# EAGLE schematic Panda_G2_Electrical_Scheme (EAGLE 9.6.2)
AUTHOR: Andrea Maroso; TITLE: Electrical Scheme

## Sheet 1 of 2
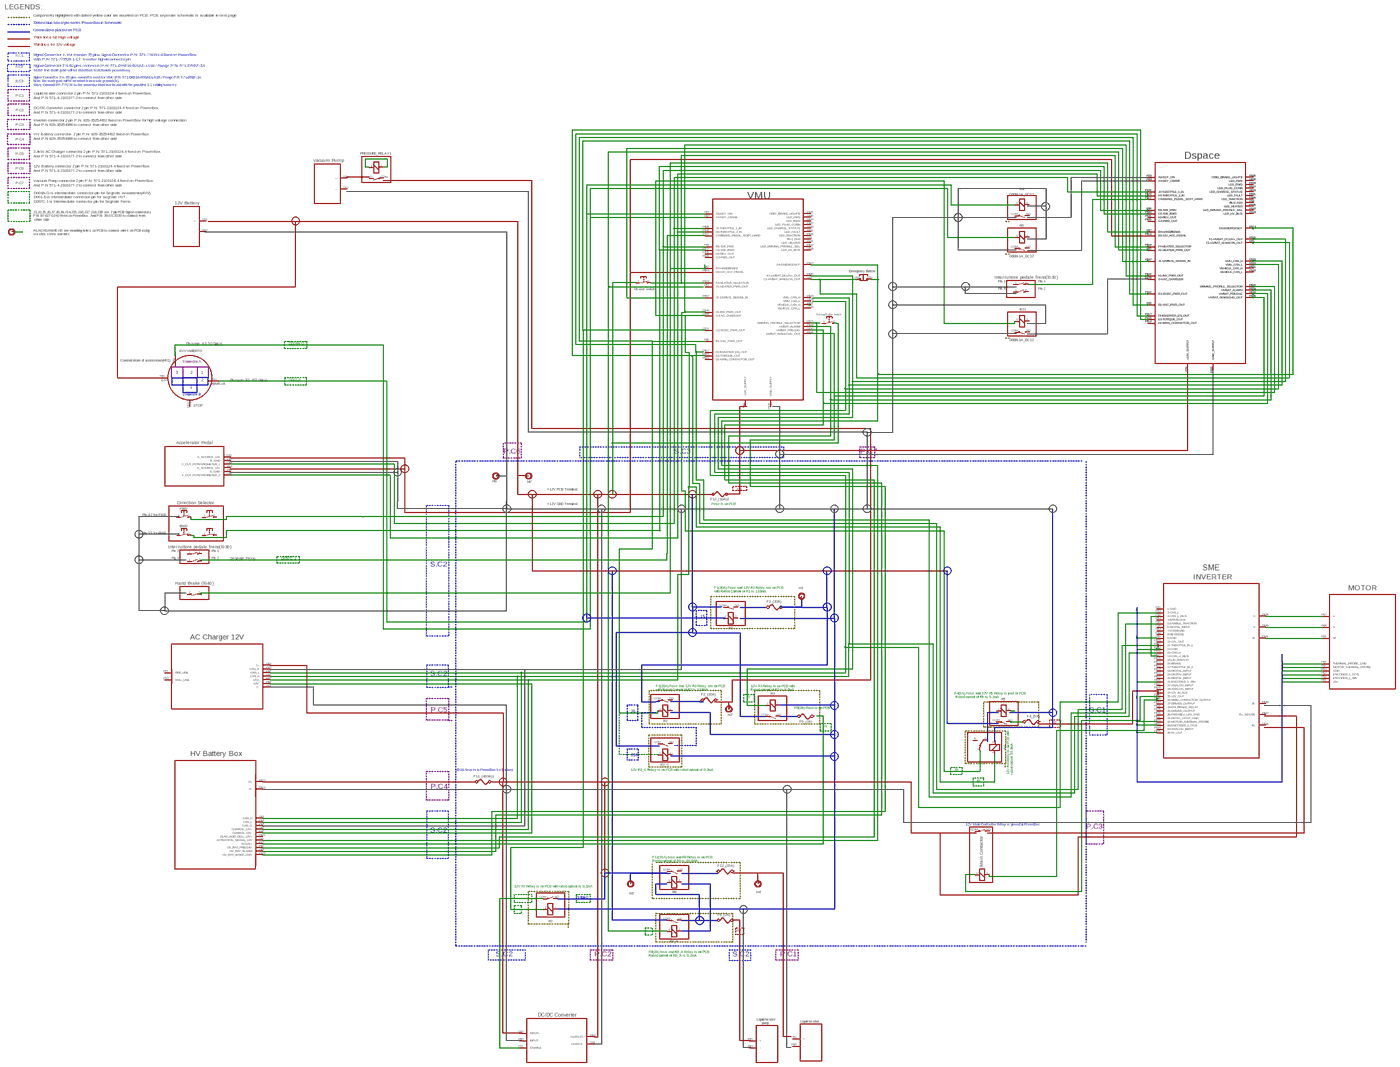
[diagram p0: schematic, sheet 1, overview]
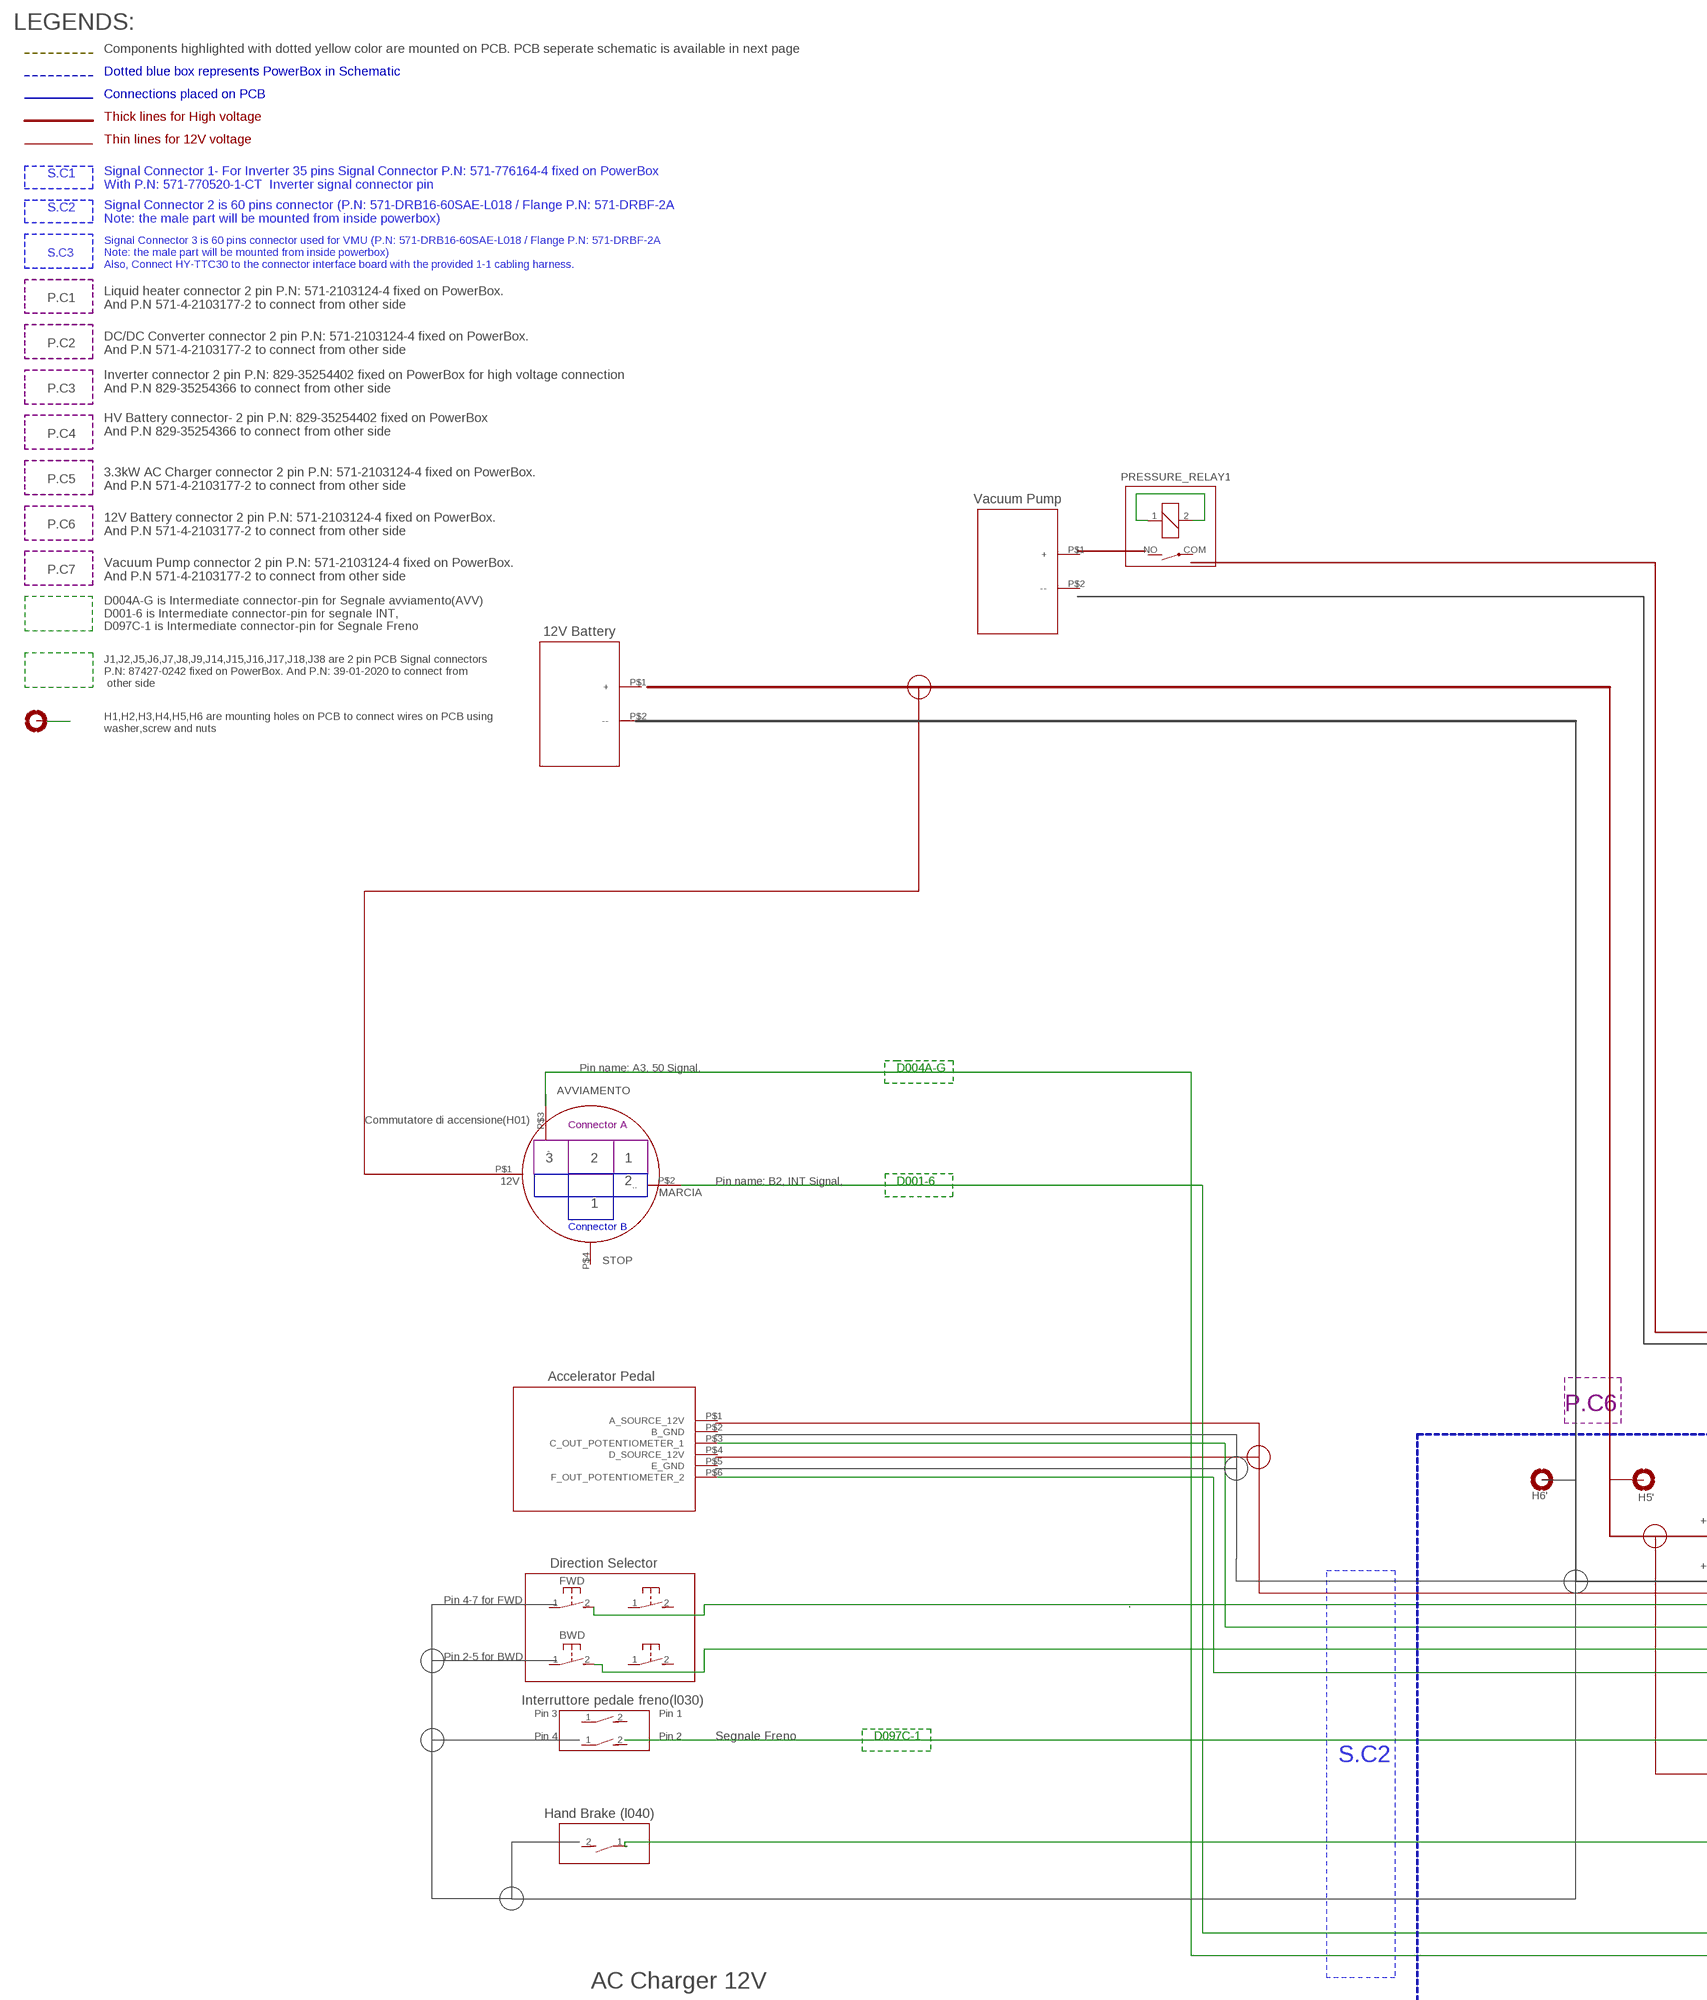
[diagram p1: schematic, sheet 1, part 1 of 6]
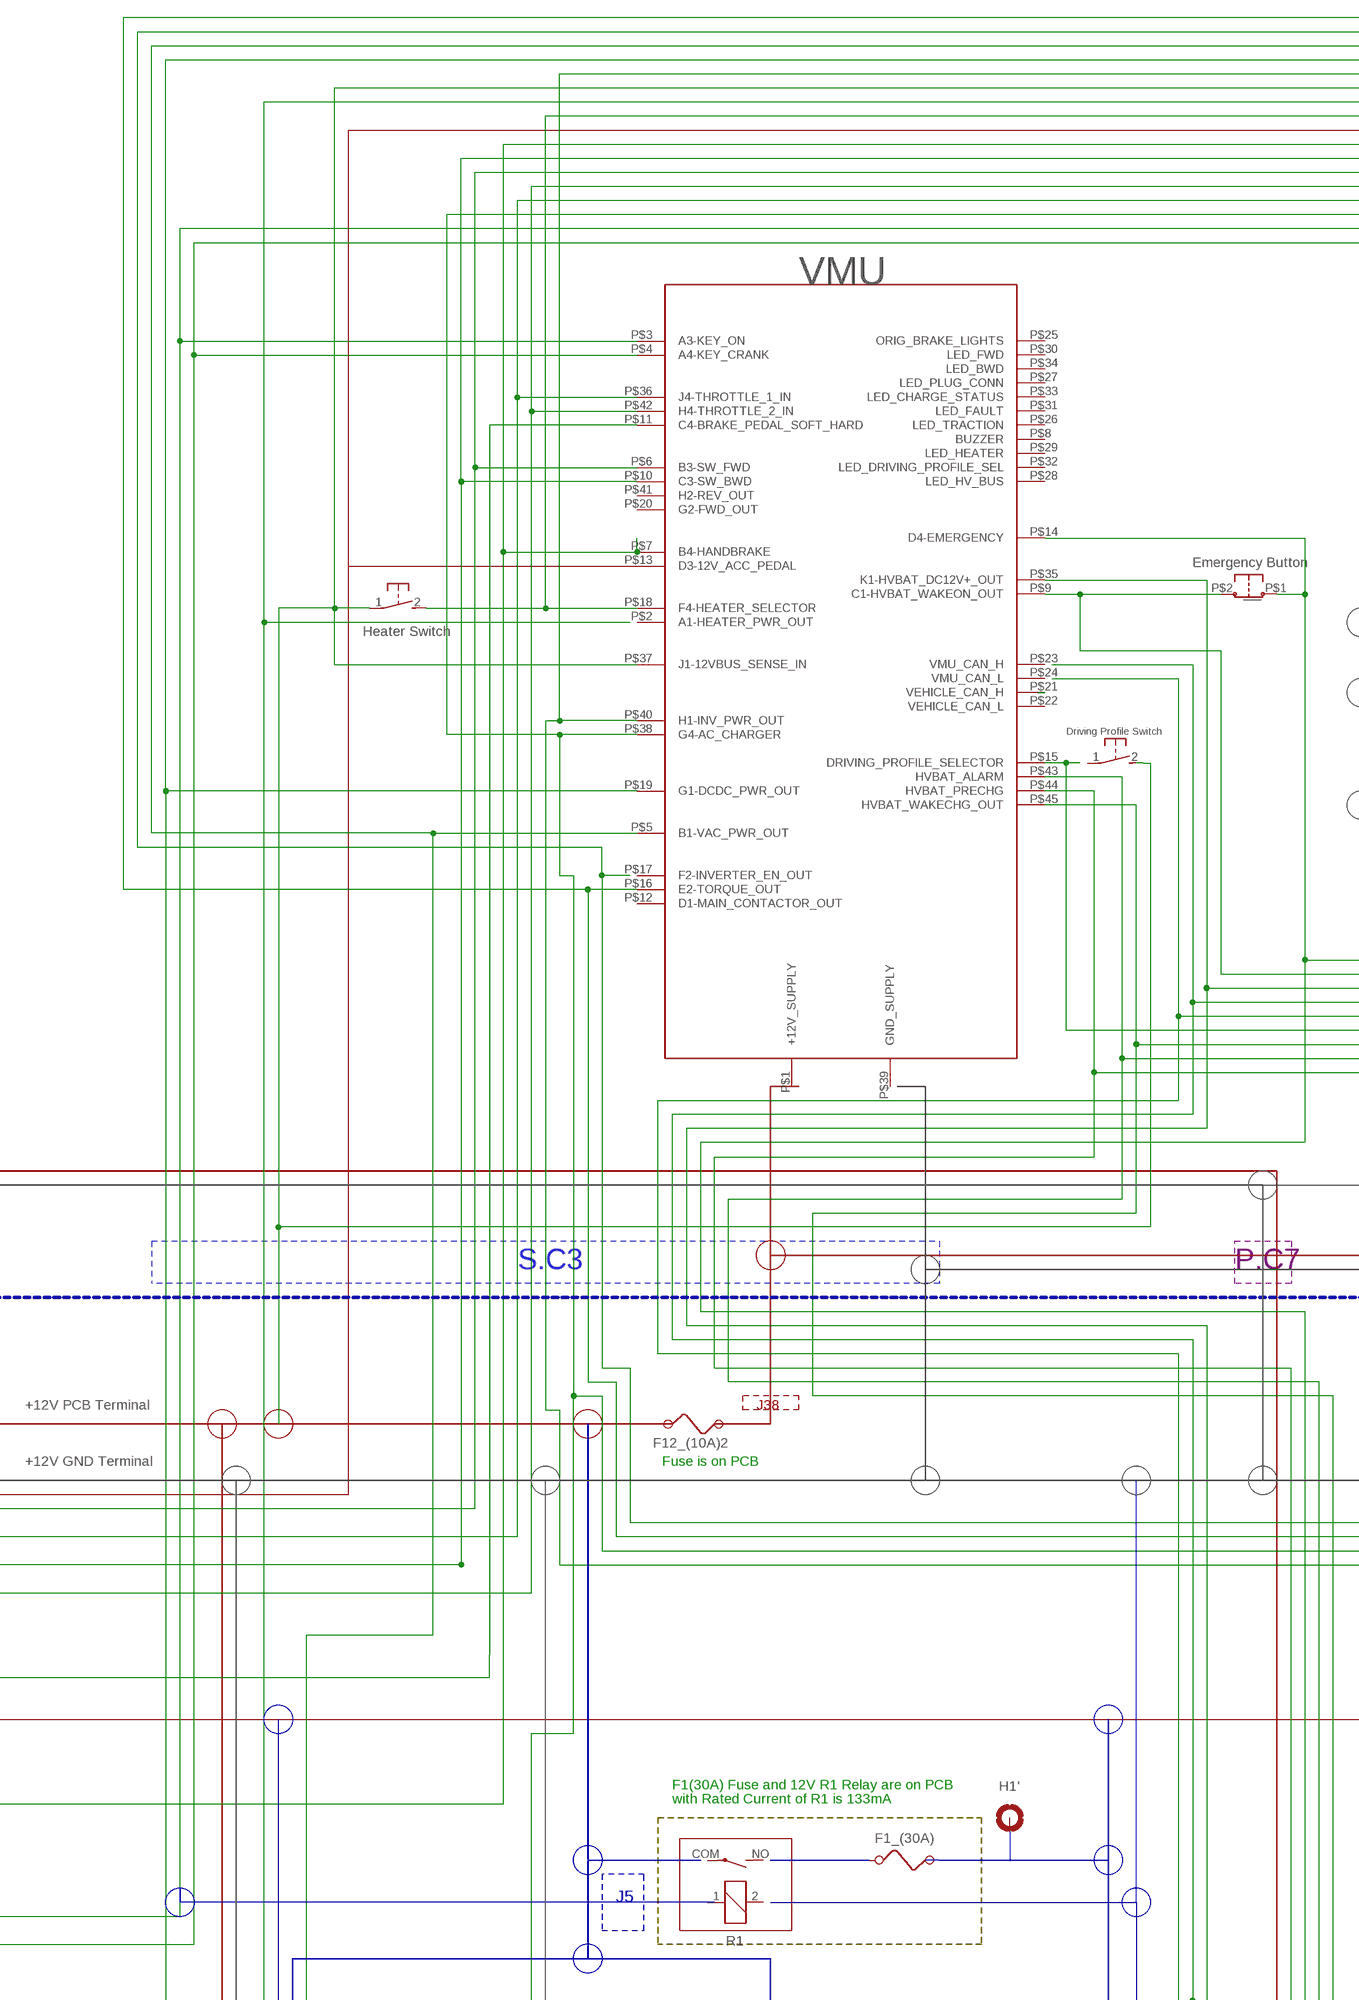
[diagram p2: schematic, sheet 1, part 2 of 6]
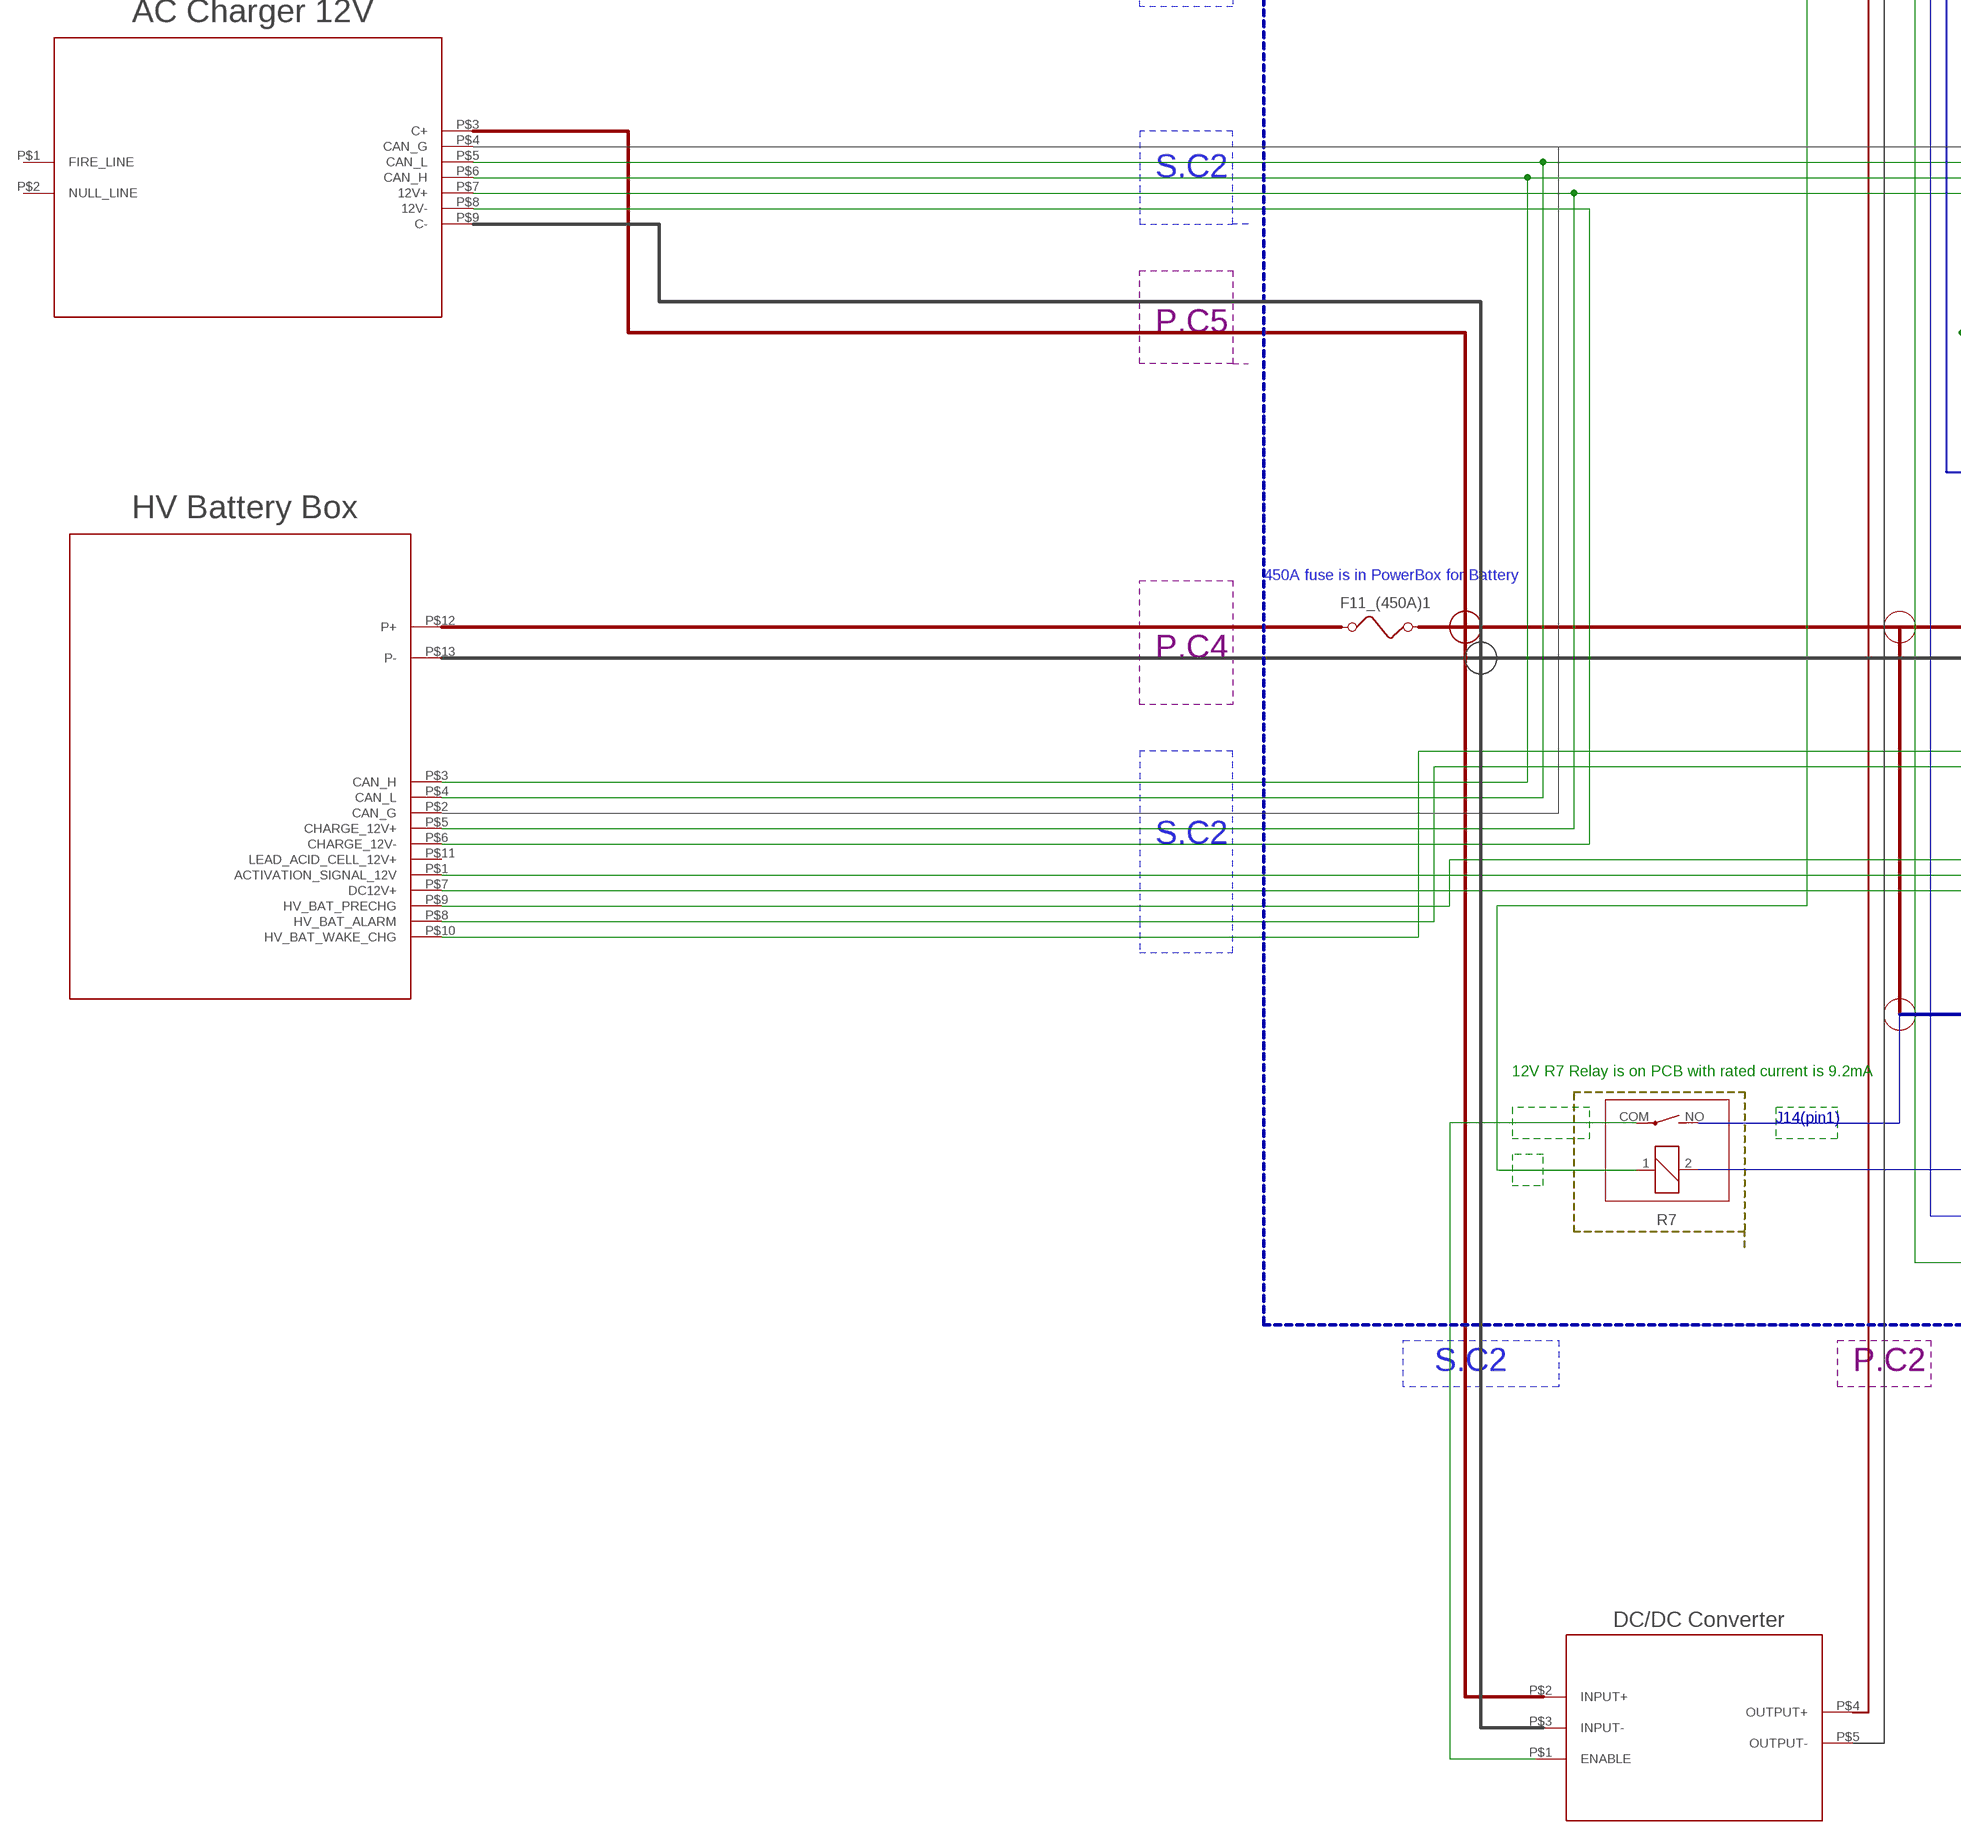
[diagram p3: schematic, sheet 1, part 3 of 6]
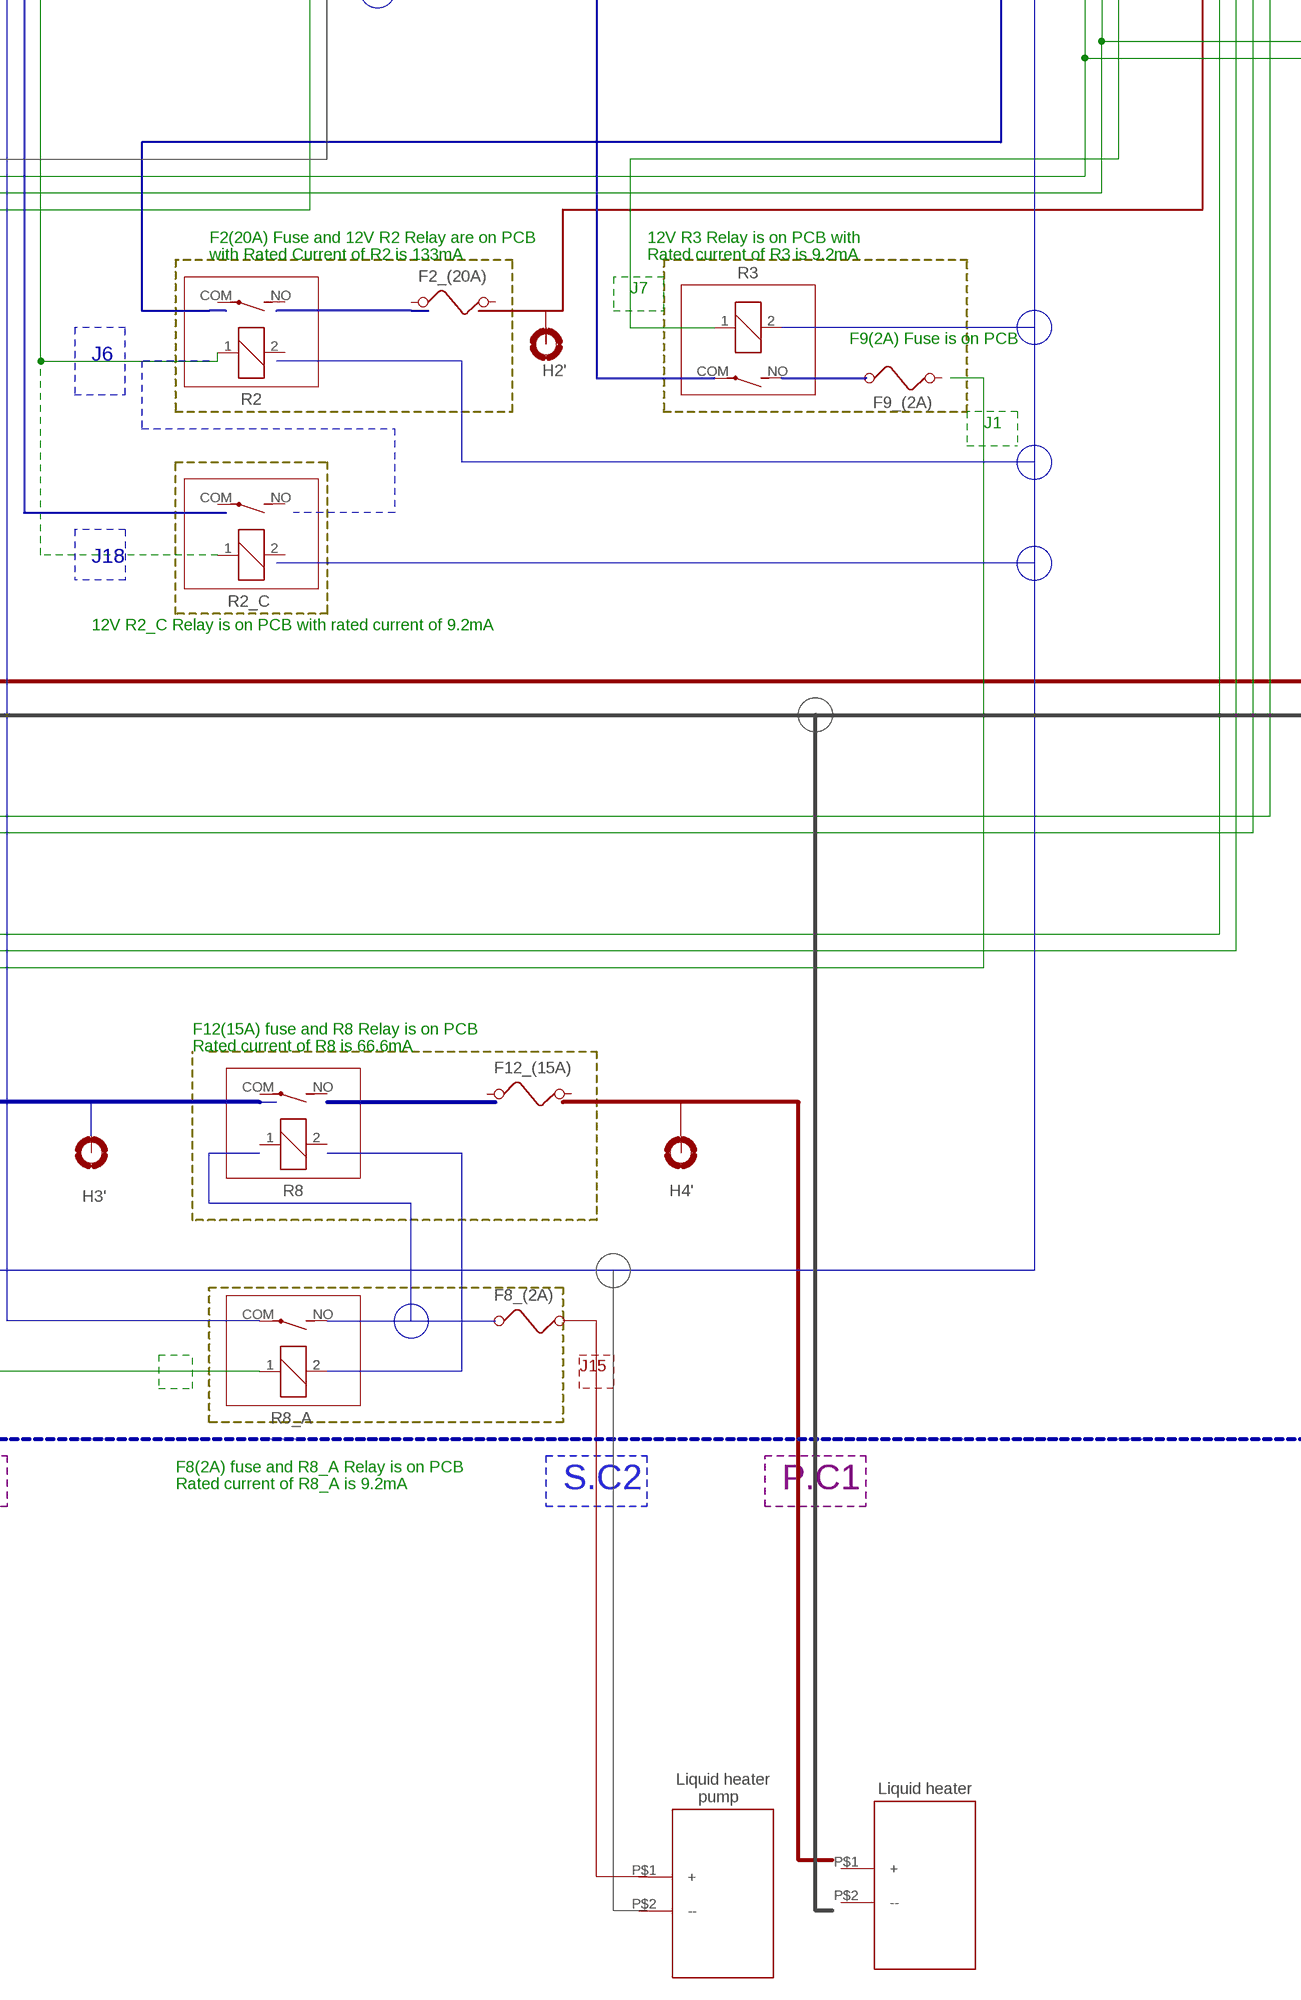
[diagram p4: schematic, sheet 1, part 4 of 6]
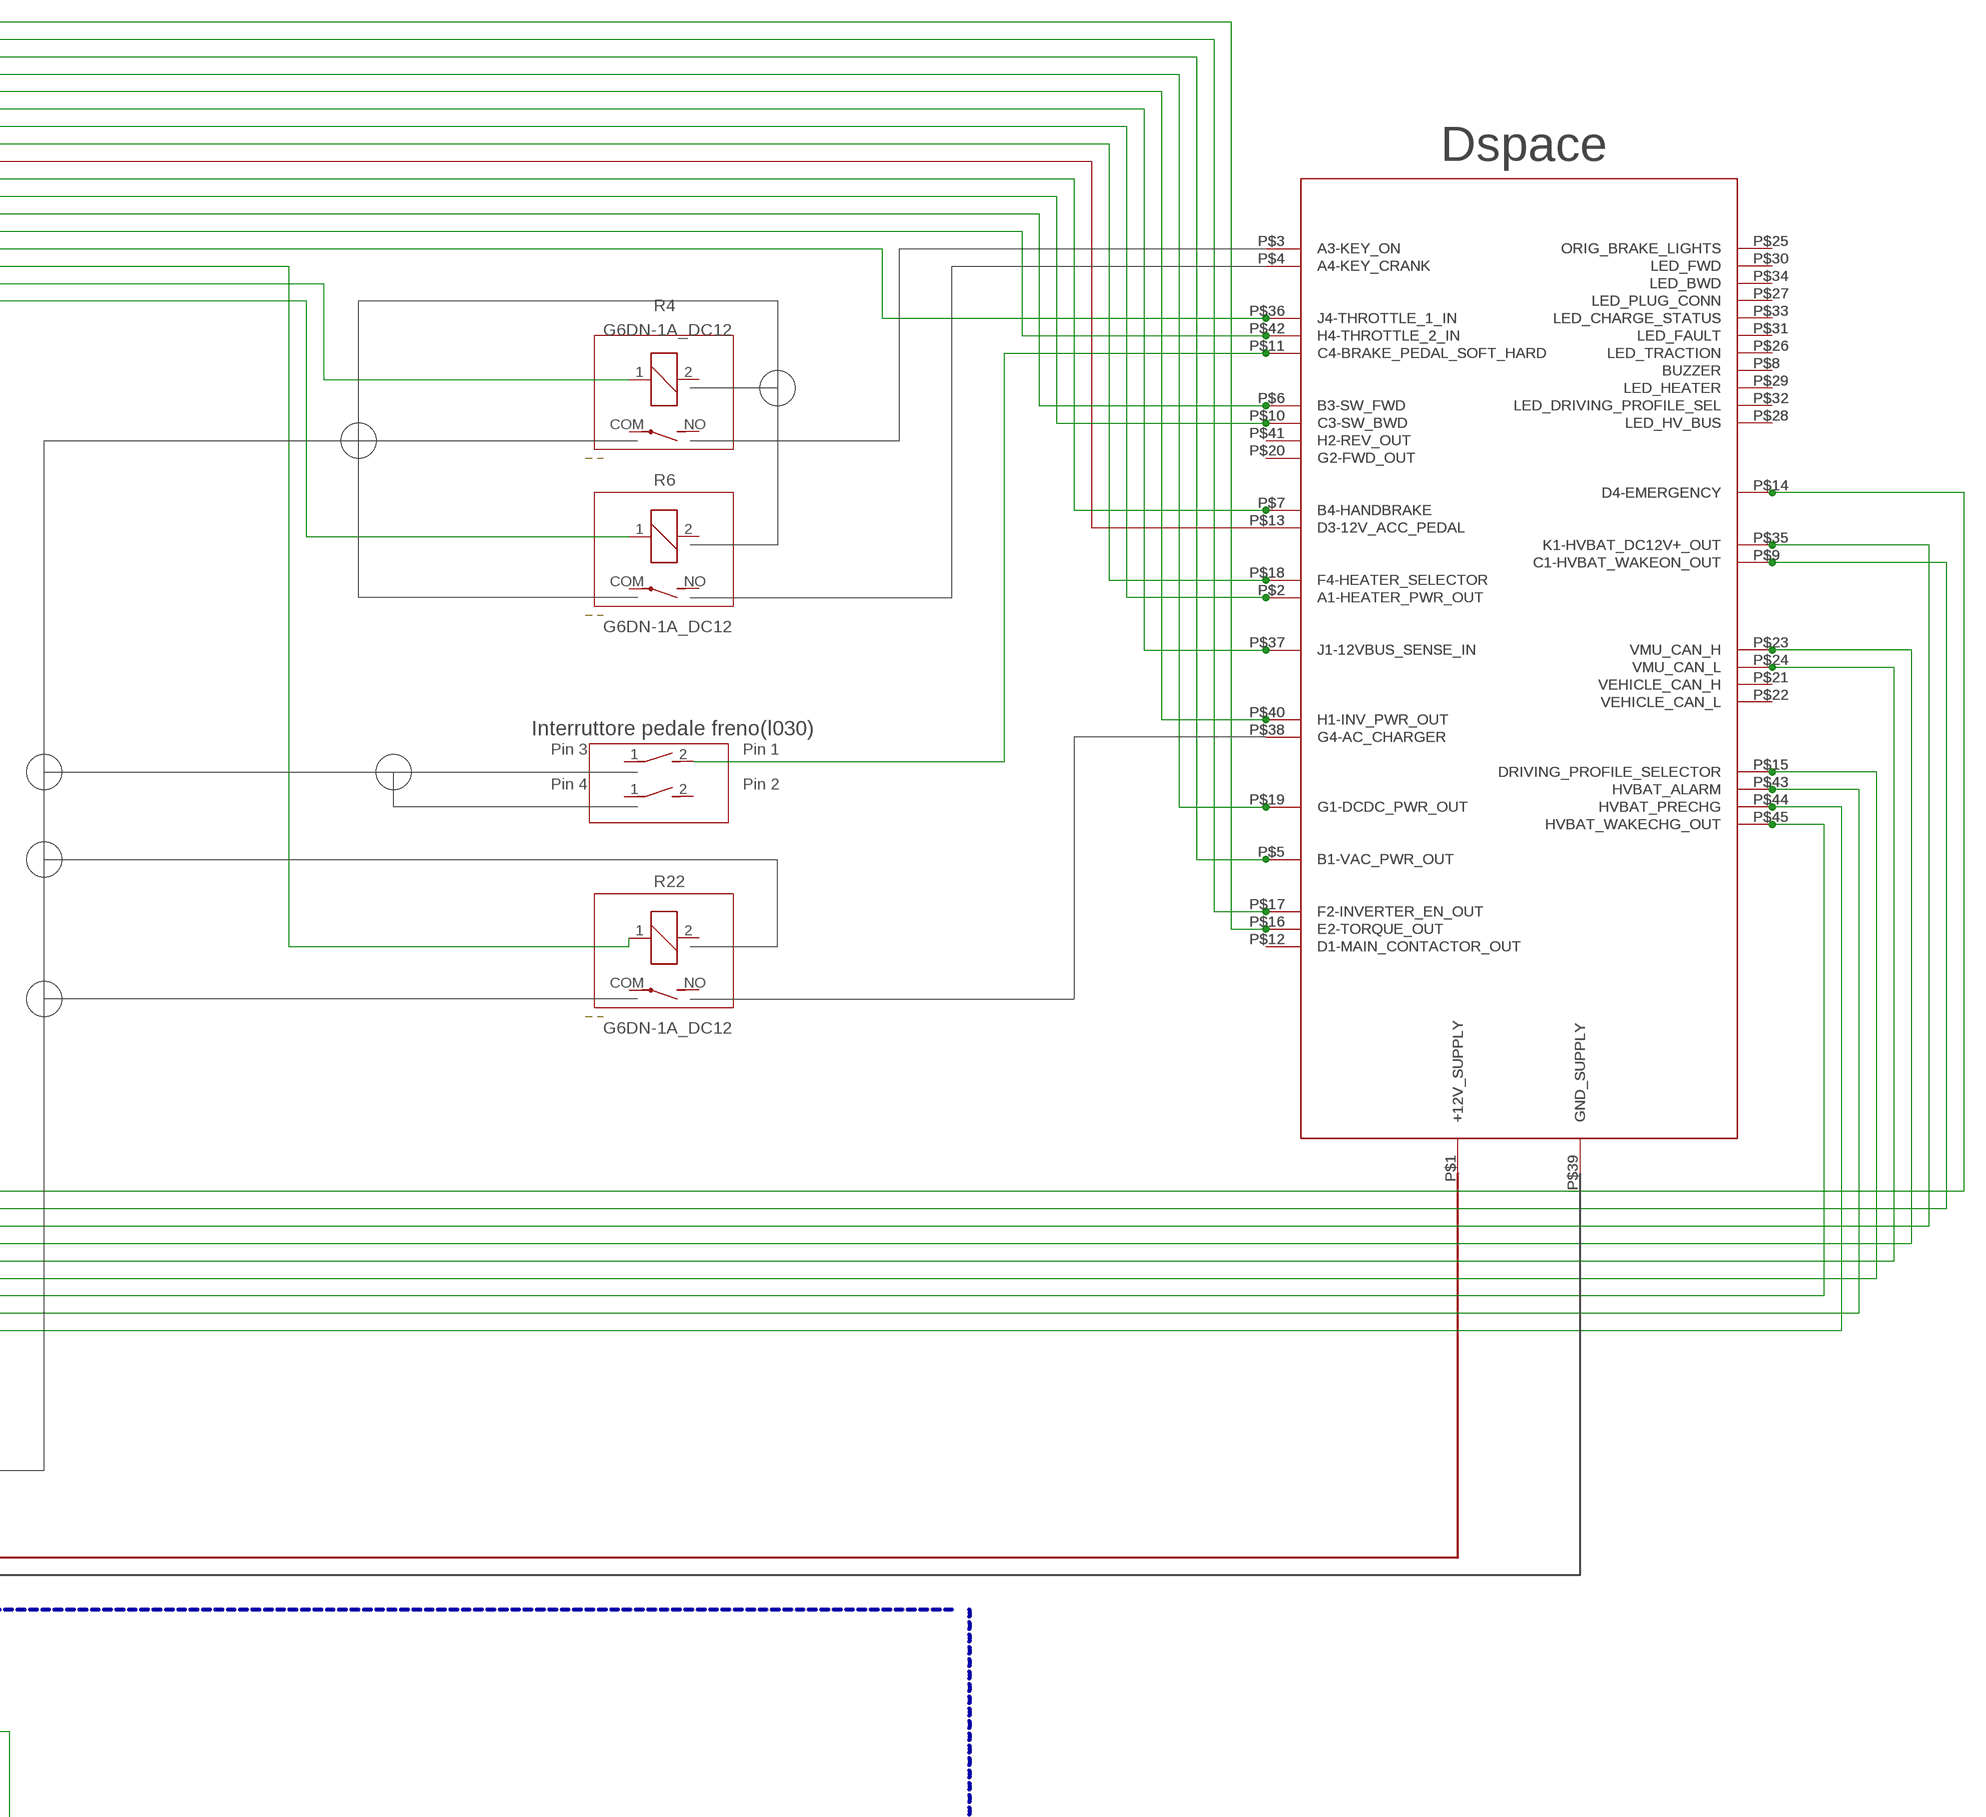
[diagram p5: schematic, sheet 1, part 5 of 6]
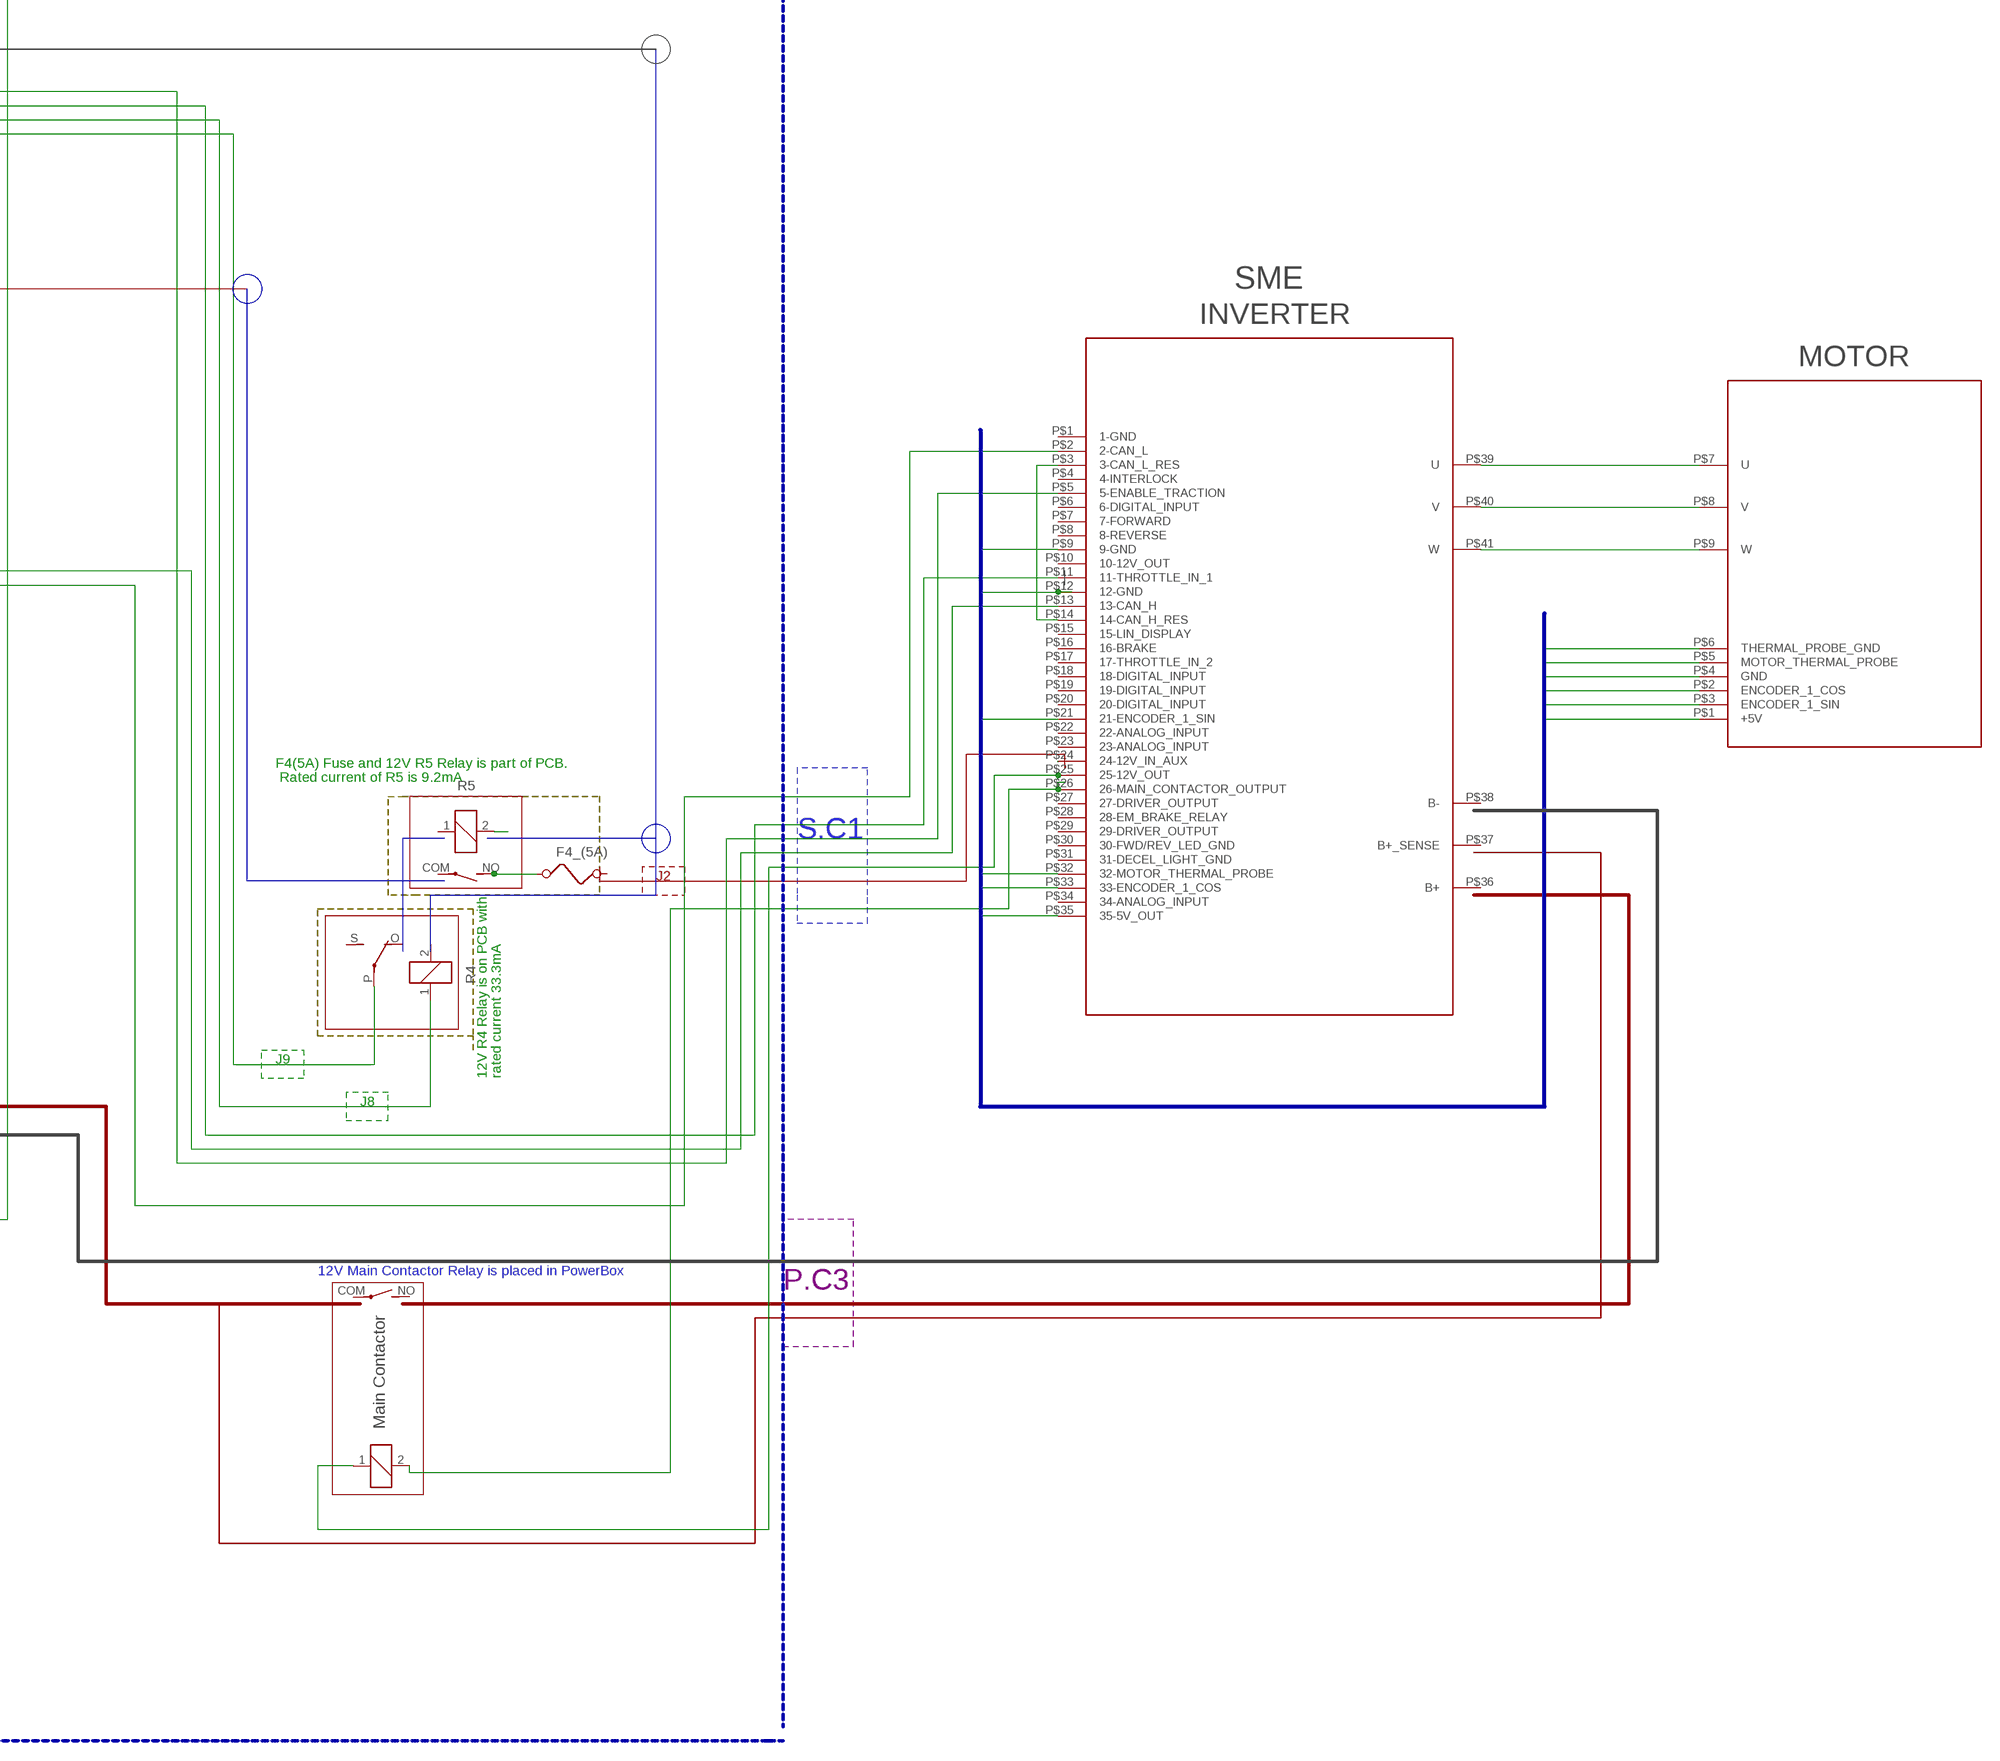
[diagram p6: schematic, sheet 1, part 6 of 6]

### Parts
DRIVING_-PROFILE_SWITCH  31-XX  [B3F-31XX]
F1_(30A)  FUSE  [FUSE]
F2_(20A)  FUSE  [FUSE]
F4_(5A)  FUSE  [FUSE]
F8_(2A)  FUSE  [FUSE]
F9_(2A)  FUSE  [FUSE]
F11_(450A)1  FUSE  [FUSE]
F12_(10A)2  FUSE  [FUSE]
F12_(15A)  FUSE  [FUSE]
H1'  MOUNT-PAD-ROUND2.25  [2,25-PAD]
H2'  MOUNT-PAD-ROUND2.25  [2,25-PAD]
H3'  MOUNT-PAD-ROUND2.25  [2,25-PAD]
H4'  MOUNT-PAD-ROUND2.25  [2,25-PAD]
H5'  MOUNT-PAD-ROUND2.25  [2,25-PAD]
H6'  MOUNT-PAD-ROUND2.25  [2,25-PAD]
H8  MOUNT-PAD-ROUND2.25  [2,25-PAD]
K2  G5L  [G5LE]
MAIN_CONTACTOR1  APF30212A  [APF30212A]
PRESSURE_RELAY1  APF30212A  [APF30212A]
R1  APF30212A  [APF30212A]
R2  APF30212A  [APF30212A]
R2_C  APF30212A  [APF30212A]
R3  APF30212A  [APF30212A]
R4  APF30212A  [APF30212A]
R5  APF30212A  [APF30212A]
R6  APF30212A  [APF30212A]
R7  APF30212A  [APF30212A]
R8  APF30212A  [APF30212A]
R8_A  APF30212A  [APF30212A]
R22  APF30212A  [APF30212A]
S1  DS01E  [DS-01]
S2  31-XX  [B3F-31XX]
S3  DS01E  [DS-01]
S4  31-XX  [B3F-31XX]
S5  31-XX  [B3F-31XX]
S6  31-XX  [B3F-31XX]
S7  DS01E  [DS-01]
S8  DS01E  [DS-01]
S9  DS01E  [DS-01]
S10  31-XX  [B3F-31XX]
U$1  IGNITION_LOCK  [IGNITION_LOCK]
U$2  EMERGENCY_BUTTON  [EMERGENCY_BUTTON]
U$3  VMU  [VMU]
U$4  VMU  [VMU]
U$14  INVERTER  [INVERTER]
U$15  MOTOR  [MOTOR]
U$16  VACUUM_PUMP  [VACUUM_PUMP]
U$19  DC/DC  [DC/DC]
U$20  LIQUID_HEATER  [LIQUID_HEATER]
U$21  LIQUID_HEATER_PUMP  [LIQUID_HEATER_PUMP]
U$22  12V_BATTERY  [12V_BATTERY]
U$23  ACC_PEDAL  [ACC_PEDAL]
U$25  HV_BATTERY_BOX  [HV_BATTERY_BOX]
U$26  1.8KW_BATTERY_CHARGER  [1.8KW_BATTERY_CHARGER]
U$27  VMU  [VMU]

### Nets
12V_GND_PCB: R5.2
+12V_PCB: DRIVING_-PROFILE_SWITCH.2(S) S10.1(P) U$3.P$37(J1-12VBUS_SENSE_IN) U$4.P$37(J1-12VBUS_SENSE_IN) U$27.P$37(J1-12VBUS_SENSE_IN)
+12VBATT1: H8.B2,25(MOUNT)
ACCHG_12V: K2.1 R22.1 U$25.P$5(CHARGE_12V+) U$26.P$7(12V+) U$27.P$38(G4-AC_CHARGER)
ACTIVATION_SIGNAL_12V: U$2.P$1(_) U$3.P$14(D4-EMERGENCY) U$4.P$14(D4-EMERGENCY) U$25.P$1(ACTIVATION_SIGNAL_12V) U$27.P$14(D4-EMERGENCY)
B$28: U$14.P$9(9-GND) U$14.P$12(12-GND) U$14.P$21(21-ENCODER_1_SIN) U$14.P$32(32-MOTOR_THERMAL_PROBE) U$14.P$33(33-ENCODER_1_COS) U$14.P$35(35-5V_OUT) U$15.P$1(+5V) U$15.P$2(ENCODER_1_COS) U$15.P$3(ENCODER_1_SIN) U$15.P$4(GND) U$15.P$5(MOTOR_THERMAL_PROBE) U$15.P$6(THERMAL_PROBE_GND)
CAN_H: U$3.P$23(VMU_CAN_H) U$4.P$23(VMU_CAN_H) U$14.P$13(13-CAN_H) U$25.P$3(CAN_H) U$26.P$6(CAN_H) U$27.P$21(VEHICLE_CAN_H)
CAN_L: U$3.P$24(VMU_CAN_L) U$4.P$24(VMU_CAN_L) U$14.P$2(2-CAN_L) U$25.P$4(CAN_L) U$26.P$5(CAN_L)
DC12V+: U$25.P$7(DC12V+)
HAND_BRAKE: S3.1 U$3.P$7(B4-HANDBRAKE) U$4.P$7(B4-HANDBRAKE) U$27.P$7(B4-HANDBRAKE)
INVERTER_PWR: K2.P(2:P) U$3.P$40(H1-INV_PWR_OUT) U$4.P$40(H1-INV_PWR_OUT) U$27.P$40(H1-INV_PWR_OUT)
N$2: R2.1 R2_C.1 U$3.P$5(B1-VAC_PWR_OUT) U$4.P$5(B1-VAC_PWR_OUT) U$27.P$5(B1-VAC_PWR_OUT)
N$3: U$3.P$44(HVBAT_PRECHG) U$4.P$44(HVBAT_PRECHG) U$25.P$9(HV_BAT_PRECHG) U$27.P$44(HVBAT_PRECHG)
N$4: U$3.P$16(E2-TORQUE_OUT) U$4.P$16(E2-TORQUE_OUT) U$14.P$11(11-THROTTLE_IN_1) U$27.P$16(E2-TORQUE_OUT)
N$5: U$3.P$17(F2-INVERTER_EN_OUT) U$4.P$17(F2-INVERTER_EN_OUT) U$14.P$5(5-ENABLE_TRACTION)
N$15: U$14.P$39(U) U$15.P$7(U)
N$18: U$14.P$40(V) U$15.P$8(V)
N$19: U$14.P$41(W) U$15.P$9(W)
N$24: U$14.P$3(3-CAN_L_RES) U$14.P$14(14-CAN_H_RES)
N$28: F9_(2A).1 R3.NO(2:S)
N$31: F4_(5A).1 R5.NO(2:S)
N$33: MAIN_CONTACTOR1.1 U$14.P$25(25-12V_OUT)
N$34: MAIN_CONTACTOR1.2 U$14.P$26(26-MAIN_CONTACTOR_OUTPUT)
N$36: PRESSURE_RELAY1.1 PRESSURE_RELAY1.2
N$37: R7.COM(2:P) U$19.P$1(ENABLE)
N$42: U$27.P$11(C4-BRAKE_PEDAL_SOFT_HARD)
N$44: S6.2(S) U$3.P$6(B3-SW_FWD) U$4.P$6(B3-SW_FWD) U$27.P$6(B3-SW_FWD)
N$46: U$3.P$36(J4-THROTTLE_1_IN) U$4.P$36(J4-THROTTLE_1_IN) U$23.P$3(C_OUT_POTENTIOMETER_1) U$27.P$36(J4-THROTTLE_1_IN)
N$47: R7.1 U$3.P$19(G1-DCDC_PWR_OUT) U$4.P$19(G1-DCDC_PWR_OUT) U$27.P$19(G1-DCDC_PWR_OUT)
N$50: U$25.P$6(CHARGE_12V-) U$26.P$8(12V-)
N$51: R3.1 U$3.P$35(K1-HVBAT_DC12V+_OUT) U$4.P$35(K1-HVBAT_DC12V+_OUT) U$27.P$35(K1-HVBAT_DC12V+_OUT)
N$52: S10.2(S) U$3.P$18(F4-HEATER_SELECTOR) U$4.P$18(F4-HEATER_SELECTOR) U$27.P$18(F4-HEATER_SELECTOR)
N$53: U$3.P$42(H4-THROTTLE_2_IN) U$4.P$42(H4-THROTTLE_2_IN) U$23.P$6(F_OUT_POTENTIOMETER_2) U$27.P$42(H4-THROTTLE_2_IN)
N$54: U$2.P$2(__) U$3.P$9(C1-HVBAT_WAKEON_OUT) U$4.P$9(C1-HVBAT_WAKEON_OUT) U$27.P$9(C1-HVBAT_WAKEON_OUT)
N$55: R4.1 U$1.P$2(..) U$27.P$3(A3-KEY_ON)
N$80: R6.1 U$1.P$3(,) U$27.P$4(A4-KEY_CRANK)
N$84: U$3.P$43(HVBAT_ALARM) U$4.P$43(HVBAT_ALARM) U$25.P$8(HV_BAT_ALARM) U$27.P$43(HVBAT_ALARM)
N$85: U$14.P$24(24-12V_IN_AUX)
N$86: U$3.P$45(HVBAT_WAKECHG_OUT) U$4.P$45(HVBAT_WAKECHG_OUT) U$25.P$10(HV_BAT_WAKE_CHG) U$27.P$45(HVBAT_WAKECHG_OUT)
N$87: U$3.P$15(DRIVING_PROFILE_SELECTOR) U$4.P$15(DRIVING_PROFILE_SELECTOR) U$27.P$15(DRIVING_PROFILE_SELECTOR)
N$88: U$3.P$21(VEHICLE_CAN_H) U$4.P$21(VEHICLE_CAN_H)
N$89: U$3.P$20(G2-FWD_OUT) U$4.P$20(G2-FWD_OUT)
N$90: U$3.P$12(D1-MAIN_CONTACTOR_OUT) U$4.P$12(D1-MAIN_CONTACTOR_OUT)
N$94: U$3.P$41(H2-REV_OUT) U$4.P$41(H2-REV_OUT)
N$98: S9.2 U$3.P$11(C4-BRAKE_PEDAL_SOFT_HARD) U$4.P$11(C4-BRAKE_PEDAL_SOFT_HARD)
N$101: U$3.P$4(A4-KEY_CRANK) U$4.P$4(A4-KEY_CRANK)
N$102: U$3.P$3(A3-KEY_ON) U$4.P$3(A3-KEY_ON)
N$107: R8_A.1 U$3.P$2(A1-HEATER_PWR_OUT) U$4.P$2(A1-HEATER_PWR_OUT)
N$110: U$3.P$1(+12V_SUPPLY) U$4.P$1(+12V_SUPPLY)
N$111: U$3.P$39(GND_SUPPLY) U$4.P$39(GND_SUPPLY)
N$112: U$3.P$13(D3-12V_ACC_PEDAL) U$4.P$13(D3-12V_ACC_PEDAL)
N$116: U$3.P$22(VEHICLE_CAN_L) U$4.P$22(VEHICLE_CAN_L)
N$117: U$3.P$38(G4-AC_CHARGER) U$4.P$38(G4-AC_CHARGER)
N$118: U$3.P$25(ORIG_BRAKE_LIGHTS) U$4.P$25(ORIG_BRAKE_LIGHTS)
N$119: U$3.P$30(LED_FWD) U$4.P$30(LED_FWD)
N$120: U$3.P$34(LED_BWD) U$4.P$34(LED_BWD)
N$121: U$3.P$27(LED_PLUG_CONN) U$4.P$27(LED_PLUG_CONN)
N$122: U$3.P$33(LED_CHARGE_STATUS) U$4.P$33(LED_CHARGE_STATUS)
N$123: U$3.P$31(LED_FAULT) U$4.P$31(LED_FAULT)
N$124: U$3.P$26(LED_TRACTION) U$4.P$26(LED_TRACTION)
N$125: U$3.P$8(BUZZER) U$4.P$8(BUZZER)
N$126: U$3.P$29(LED_HEATER) U$4.P$29(LED_HEATER)
N$127: U$3.P$32(LED_DRIVING_PROFILE_SEL) U$4.P$32(LED_DRIVING_PROFILE_SEL)
N$128: U$3.P$28(LED_HV_BUS) U$4.P$28(LED_HV_BUS)
REV1: S2.2(S) U$3.P$10(C3-SW_BWD) U$4.P$10(C3-SW_BWD) U$27.P$10(C3-SW_BWD)
Unconnected: DRIVING_-PROFILE_SWITCH.1(P) F1_(30A).1 F1_(30A).2 F2_(20A).1 F2_(20A).2 F4_(5A).2 F8_(2A).1 F8_(2A).2 F9_(2A).2 F11_(450A)1.1 F11_(450A)1.2 F12_(10A)2.1 F12_(10A)2.2 F12_(15A).1 F12_(15A).2 H1'.B2,25(MOUNT) H2'.B2,25(MOUNT) H3'.B2,25(MOUNT) H4'.B2,25(MOUNT) H5'.B2,25(MOUNT) H6'.B2,25(MOUNT) K2.2 K2.O(2:O) K2.S(2:S) MAIN_CONTACTOR1.COM(2:P) MAIN_CONTACTOR1.NO(2:S) PRESSURE_RELAY1.COM(2:P) PRESSURE_RELAY1.NO(2:S) R1.1 R1.2 R1.COM(2:P) R1.NO(2:S) R2.2 R2.COM(2:P) R2.NO(2:S) R2_C.2 R2_C.COM(2:P) R2_C.NO(2:S) R3.2 R3.COM(2:P) R4.2 R4.COM(2:P) R4.NO(2:S) R5.1 R5.COM(2:P) R6.2 R6.COM(2:P) R6.NO(2:S) R7.2 R7.NO(2:S) R8.1 R8.2 R8.COM(2:P) R8.NO(2:S) R8_A.2 R8_A.COM(2:P) R8_A.NO(2:S) R22.2 R22.COM(2:P) R22.NO(2:S) S1.1 S1.2 S2.1(P) S3.2 S4.1(P) S4.2(S) S5.1(P) S5.2(S) S6.1(P) S7.1 S7.2 S8.1 S8.2 S9.1 U$1.P$1(.) U$1.P$4(') U$14.P$1(1-GND) U$14.P$4(4-INTERLOCK) U$14.P$6(6-DIGITAL_INPUT) U$14.P$7(7-FORWARD) U$14.P$8(8-REVERSE) U$14.P$10(10-12V_OUT) U$14.P$15(15-LIN_DISPLAY) U$14.P$16(16-BRAKE) U$14.P$17(17-THROTTLE_IN_2) U$14.P$18(18-DIGITAL_INPUT) U$14.P$19(19-DIGITAL_INPUT) U$14.P$20(20-DIGITAL_INPUT) U$14.P$22(22-ANALOG_INPUT) U$14.P$23(23-ANALOG_INPUT) U$14.P$27(27-DRIVER_OUTPUT) U$14.P$28(28-EM_BRAKE_RELAY) U$14.P$29(29-DRIVER_OUTPUT) U$14.P$30(30-FWD/REV_LED_GND) U$14.P$31(31-DECEL_LIGHT_GND) U$14.P$34(34-ANALOG_INPUT) U$14.P$36(B+) U$14.P$37(B+_SENSE) U$14.P$38(B-) U$16.P$1(+) U$16.P$2(--) U$19.P$2(INPUT+) U$19.P$3(INPUT-) U$19.P$4(OUTPUT+) U$19.P$5(OUTPUT-) U$20.P$1(+) U$20.P$2(--) U$21.P$1(+) U$21.P$2(--) U$22.P$1(+) U$22.P$2(--) U$23.P$1(A_SOURCE_12V) U$23.P$2(B_GND) U$23.P$4(D_SOURCE_12V) U$23.P$5(E_GND) U$25.P$2(CAN_G) U$25.P$11(LEAD_ACID_CELL_12V+) U$26.P$1(FIRE_LINE) U$26.P$2(NULL_LINE) U$26.P$3(C+) U$26.P$4(CAN_G) U$26.P$9(C-) U$27.P$1(+12V_SUPPLY) U$27.P$2(A1-HEATER_PWR_OUT) U$27.P$8(BUZZER) U$27.P$12(D1-MAIN_CONTACTOR_OUT) U$27.P$13(D3-12V_ACC_PEDAL) U$27.P$17(F2-INVERTER_EN_OUT) U$27.P$20(G2-FWD_OUT) U$27.P$22(VEHICLE_CAN_L) U$27.P$23(VMU_CAN_H) U$27.P$24(VMU_CAN_L) U$27.P$25(ORIG_BRAKE_LIGHTS) U$27.P$26(LED_TRACTION) U$27.P$27(LED_PLUG_CONN) U$27.P$28(LED_HV_BUS) U$27.P$29(LED_HEATER) U$27.P$30(LED_FWD) U$27.P$31(LED_FAULT) U$27.P$32(LED_DRIVING_PROFILE_SEL) U$27.P$33(LED_CHARGE_STATUS) U$27.P$34(LED_BWD) U$27.P$39(GND_SUPPLY) U$27.P$41(H2-REV_OUT)

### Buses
B$1
B$2
B$3
B$4
B$5
B$6
B$7
B$8
B$9
B$10
B$11
B$12
B$13
B$15
B$16
B$17
B$18
B$19
B$20
B$21
B$14
B$22
B$23
B$24
B$25
B$26
B$27
B$28

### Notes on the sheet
- LEGENDS:
- Components highlighted with dotted yellow color are mounted on PCB. PCB seperate schematic is available in next page
- Dotted blue box represents PowerBox in Schematic
- Connections placed on PCB
- Thick lines for High voltage
- Thin lines for 12V voltage
- S.C1
- Signal Connector 1- For Inverter 35 pins Signal Connector P.N: 571-776164-4 fixed on PowerBox
  With P.N: 571-770520-1-CT  Inverter signal connector pin
- S.C2
- Signal Connector 2 is 60 pins connector (P.N: 571-DRB16-60SAE-L018 / Flange P.N: 571-DRBF-2A 
  Note: the male part will be mounted from inside powerbox)
- S.C3
- Signal Connector 3 is 60 pins connector used for VMU (P.N: 571-DRB16-60SAE-L018 / Flange P.N: 571-DRBF-2A 
  Note: the male part will be mounted from inside powerbox)
  Also, Connect HY-TTC30 to the connector interface board with the provided 1-1 cabling harness.
- P.C1
- Liquid heater connector 2 pin P.N: 571-2103124-4 fixed on PowerBox.
  And P.N 571-4-2103177-2 to connect from other side
- P.C2
- DC/DC Converter connector 2 pin P.N: 571-2103124-4 fixed on PowerBox.
  And P.N 571-4-2103177-2 to connect from other side
- P.C3
- Inverter connector 2 pin P.N: 829-35254402 fixed on PowerBox for high voltage connection
  And P.N 829-35254366 to connect from other side
- P.C4
- HV Battery connector- 2 pin P.N: 829-35254402 fixed on PowerBox 
  And P.N 829-35254366 to connect from other side
- P.C5
- Dspace
- 3.3kW AC Charger connector 2 pin P.N: 571-2103124-4 fixed on PowerBox.
  And P.N 571-4-2103177-2 to connect from other side
- P.C6
- 12V Battery connector 2 pin P.N: 571-2103124-4 fixed on PowerBox.
  And P.N 571-4-2103177-2 to connect from other side
- P.C7
- Vacuum Pump connector 2 pin P.N: 571-2103124-4 fixed on PowerBox.
  And P.N 571-4-2103177-2 to connect from other side
- G6DN-1A_DC12
- VMU
- D004A-G is Intermediate connector-pin for Segnale avviamento(AVV)
  D001-6 is Intermediate connector-pin for segnale INT,
  D097C-1 is Intermediate connector-pin for Segnale Freno
- J1,J2,J5,J6,J7,J8,J9,J14,J15,J16,J17,J18,J38 are 2 pin PCB Signal connectors 
  P.N: 87427-0242 fixed on PowerBox. And P.N: 39-01-2020 to connect from
   other side
- H1,H2,H3,H4,H5,H6 are mounting holes on PCB to connect wires on PCB using 
  washer,screw and nuts
- G6DN-1A_DC12
- Interruttore pedale freno(l030)
- Pin 3 | Pin 1
- Heater Switch | Pin 4 | Pin 2
- Driving Profile Switch
- G6DN-1A_DC12
- Pin name: A3, 50 Signal, | D004A-G
- AVVIAMENTO
- 12V | Pin name: B2, INT Signal, | D001-6
- MARCIA
- STOP
- P.C6 | S.C3 | P.C7
- +12V PCB Terminal | J38
- Direction Selector | +12V GND Terminal | Fuse is on PCB
- FWD
- Pin 4-7 for FWD
- BWD
- Pin 2-5 for BWD
- Interruttore pedale freno(l030)
- Pin 3 | Pin 1
- Pin 4 | Pin 2 | Segnale Freno | D097C-1
- S.C2
- SME
- Hand Brake (l040)
- F1(30A) Fuse and 12V R1 Relay are on PCB
- with Rated Current of R1 is 133mA
- J5
- S.C2
- F2(20A) Fuse and 12V R2 Relay are on PCB | 12V R3 Relay is on PCB with
- with Rated Current of R2 is 133mA | Rated current of R3 is 9.2mA
- F4(5A) Fuse and 12V R5 Relay is part of PCB.
- J7 | Rated current of R5 is 9.2mA
- F9(2A) Fuse is on PCB
- P.C5 | J6 | S.C1
- J2
- J1
- R4
- J18
- 450A fuse is in PowerBox for Battery | 12V R2_C Relay is on PCB with rated current of 9.2mA | J9
- 12V R4 Relay is on PCB with | rated current 33.3mA
- J8
- P.C4
- 12V Main Contactor Relay is placed in PowerBox
- P.C3
- S.C2
- Main Contactor
- F12(15A) fuse and R8 Relay is on PCB
- Rated current of R8 is 66.6mA
- 12V R7 Relay is on PCB with rated current is 9.2mA
- J14(pin2) | J14(pin1)
- J16
- J17 | J15
- F8(2A) fuse and R8_A Relay is on PCB
- S.C2 | P.C2 | Rated current of R8_A is 9.2mA | S.C2 | P.C1

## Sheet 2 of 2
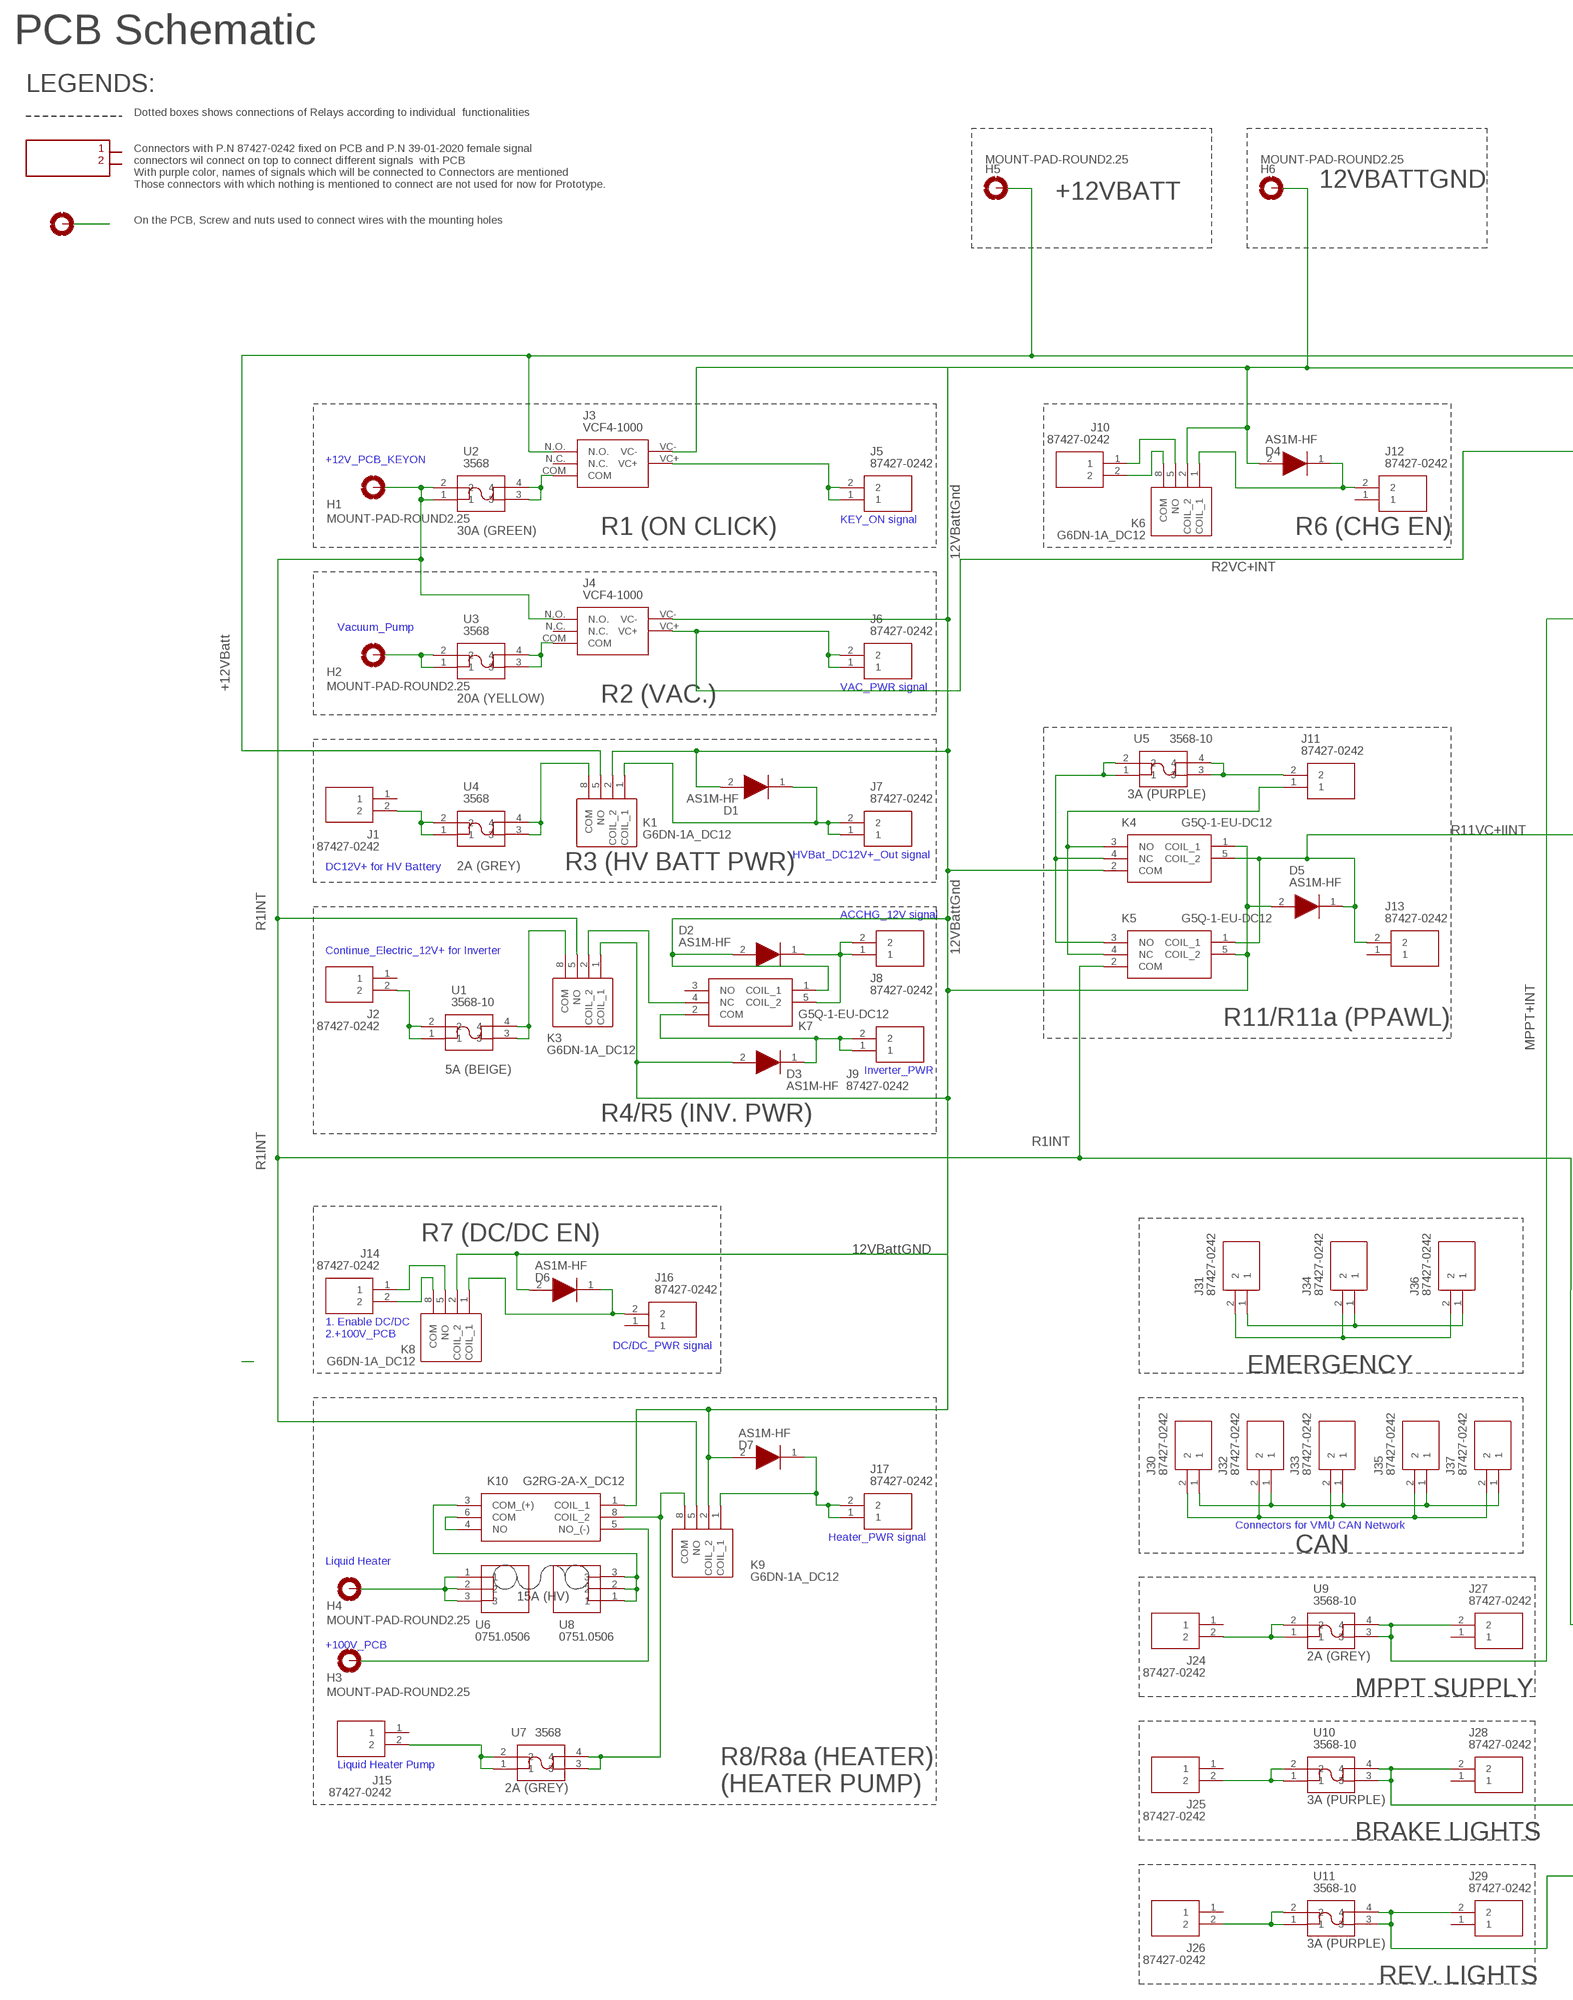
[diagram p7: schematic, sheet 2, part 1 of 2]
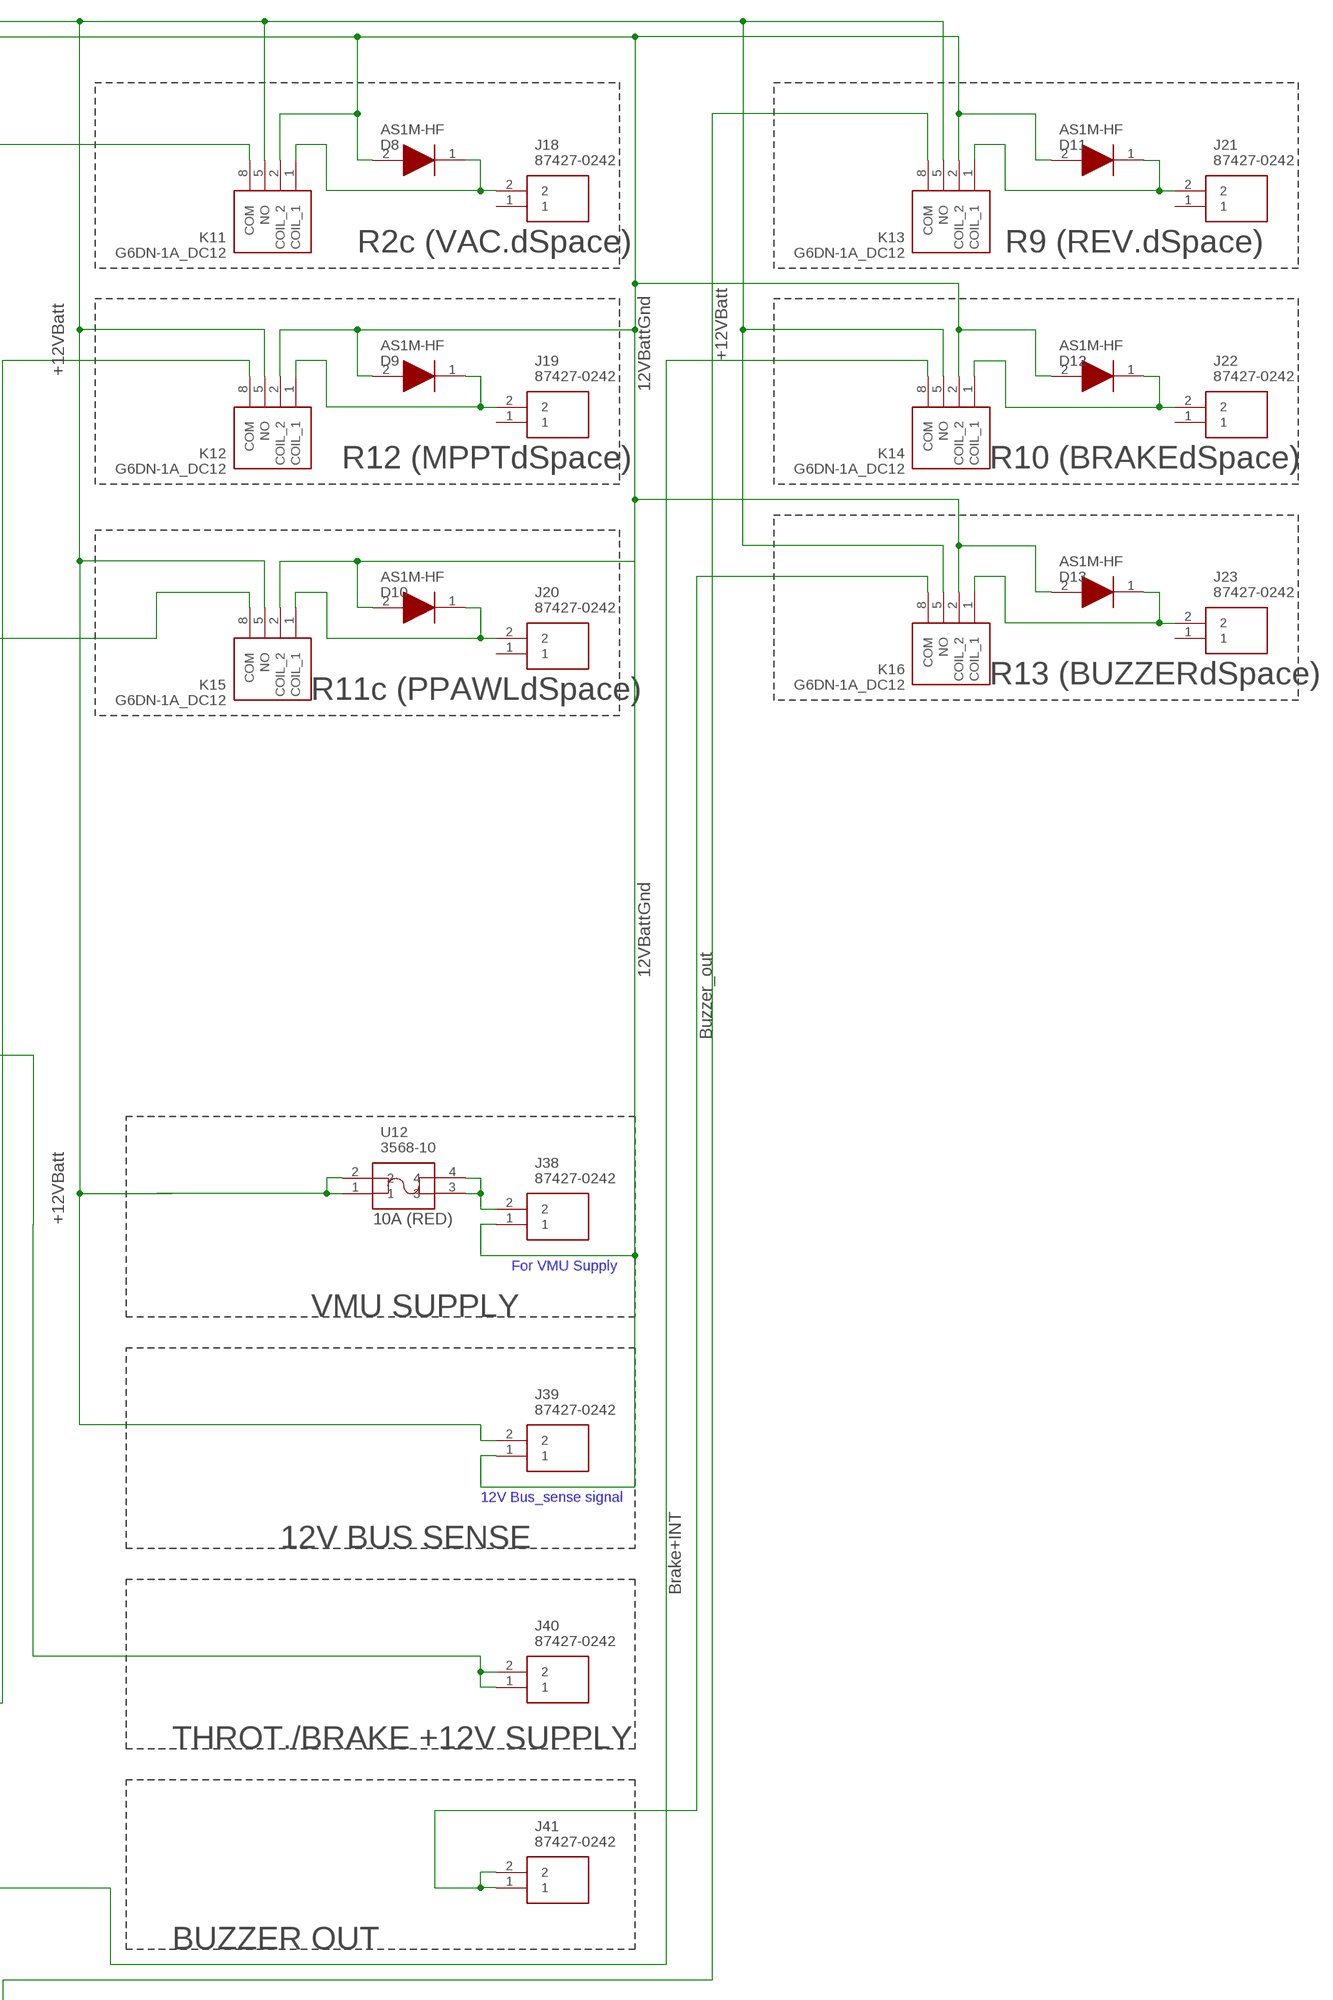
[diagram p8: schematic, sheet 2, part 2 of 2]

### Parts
D1  AS1M-HF  [DIOM5126X215N]
D2  AS1M-HF  [DIOM5126X215N]
D3  AS1M-HF  [DIOM5126X215N]
D4  AS1M-HF  [DIOM5126X215N]
D5  AS1M-HF  [DIOM5126X215N]
D6  AS1M-HF  [DIOM5126X215N]
D7  AS1M-HF  [DIOM5126X215N]
D8  AS1M-HF  [DIOM5126X215N]
D9  AS1M-HF  [DIOM5126X215N]
D10  AS1M-HF  [DIOM5126X215N]
D11  AS1M-HF  [DIOM5126X215N]
D12  AS1M-HF  [DIOM5126X215N]
D13  AS1M-HF  [DIOM5126X215N]
H1  MOUNT-PAD-ROUND2.25  [2,25-PAD]
H2  MOUNT-PAD-ROUND2.25  [2,25-PAD]
H3  MOUNT-PAD-ROUND2.25  [2,25-PAD]
H4  MOUNT-PAD-ROUND2.25  [2,25-PAD]
H5  MOUNT-PAD-ROUND2.25  [2,25-PAD]
H6  MOUNT-PAD-ROUND2.25  [2,25-PAD]
H7  MOUNT-PAD-ROUND2.25  [2,25-PAD]
J1  87427-0242  [874270242]
J2  87427-0242  [874270242]
J3  VCF4-1000  [VCF4-1000]
J4  VCF4-1000  [VCF4-1000]
J5  87427-0242  [874270242]
J6  87427-0242  [874270242]
J7  87427-0242  [874270242]
J8  87427-0242  [874270242]
J9  87427-0242  [874270242]
J10  87427-0242  [874270242]
J11  87427-0242  [874270242]
J12  87427-0242  [874270242]
J13  87427-0242  [874270242]
J14  87427-0242  [874270242]
J15  87427-0242  [874270242]
J16  87427-0242  [874270242]
J17  87427-0242  [874270242]
J18  87427-0242  [874270242]
J19  87427-0242  [874270242]
J20  87427-0242  [874270242]
J21  87427-0242  [874270242]
J22  87427-0242  [874270242]
J23  87427-0242  [874270242]
J24  87427-0242  [874270242]
J25  87427-0242  [874270242]
J26  87427-0242  [874270242]
J27  87427-0242  [874270242]
J28  87427-0242  [874270242]
J29  87427-0242  [874270242]
J30  87427-0242  [874270242]
J31  87427-0242  [874270242]
J32  87427-0242  [874270242]
J33  87427-0242  [874270242]
J34  87427-0242  [874270242]
J35  87427-0242  [874270242]
J36  87427-0242  [874270242]
J37  87427-0242  [874270242]
J38  87427-0242  [874270242]
J39  87427-0242  [874270242]
J40  87427-0242  [874270242]
J41  87427-0242  [874270242]
K1  G6DN-1A_DC12  [G6DN1ADC12]
K3  G6DN-1A_DC12  [G6DN1ADC12]
K4  G5Q-1-EU-DC12  [G5Q1EUDC12]
K5  G5Q-1-EU-DC12  [G5Q1EUDC12]
K6  G6DN-1A_DC12  [G6DN1ADC12]
K7  G5Q-1-EU-DC12  [G5Q1EUDC12]
K8  G6DN-1A_DC12  [G6DN1ADC12]
K9  G6DN-1A_DC12  [G6DN1ADC12]
K10  G2RG-2A-X_DC12  [G2RG2AXDC12]
K11  G6DN-1A_DC12  [G6DN1ADC12]
K12  G6DN-1A_DC12  [G6DN1ADC12]
K13  G6DN-1A_DC12  [G6DN1ADC12]
K14  G6DN-1A_DC12  [G6DN1ADC12]
K15  G6DN-1A_DC12  [G6DN1ADC12]
K16  G6DN-1A_DC12  [G6DN1ADC12]
U1  3568-10  [356810]
U2  3568  [3568]
U3  3568  [3568]
U4  3568  [3568]
U5  3568-10  [356810]
U6  0751.0506  [07510506]
U7  3568  [3568]
U8  0751.0506  [07510506]
U9  3568-10  [356810]
U10  3568-10  [356810]
U11  3568-10  [356810]
U12  3568-10  [356810]

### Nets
12VBATTGND: D1.2(A) D2.2(A) D3.2(A) D4.2(A) D5.2(A) D6.2(A) D7.2(A) D8.2(A) D9.2(A) D10.2(A) D11.2(A) D12.2(A) D13.2(A) H6.B2,25(MOUNT) J3.VC- J4.VC- J38.1 J39.1 K1.2(COIL_2) K3.1(COIL_1) K4.1(COIL_1) K4.2(COM) K5.5(COIL_2) K6.2(COIL_2) K7.1(COIL_1) K8.2(COIL_2) K9.2(COIL_2) K10.1(COIL_1) K11.2(COIL_2) K12.2(COIL_2) K13.2(COIL_2) K14.2(COIL_2) K15.2(COIL_2) K16.2(COIL_2)
+12VBATT: H5.B2,25(MOUNT) J3.N.O. J39.2 K1.5(NO) K11.5(NO) K12.5(NO) K13.5(NO) K14.5(NO) K15.5(NO) K16.5(NO) U12.1 U12.2
BRAKE+INT: J28.2 K14.8(COM) U10.3 U10.4
BUZZER_OUT: J41.1 J41.2 K16.8(COM)
CAN_N [CAN diff]: J30.1 J32.1 J33.1 J35.1 J37.1
CAN_P [CAN diff]: J30.2 J32.2 J33.2 J35.2 J37.2
MPPT+INT: J27.2 K12.8(COM) U9.3 U9.4
N$8: J3.COM U2.3 U2.4
N$9: J4.COM U3.3 U3.4
N$10: H2.B2,25(MOUNT) U3.1 U3.2
N$11: J3.VC+ J5.1 J5.2
N$12: K1.8(COM) U4.3 U4.4
N$13: J1.2 U4.1 U4.2
N$14: D1.1(K) J7.1 J7.2 K1.1(COIL_1)
N$16: J2.2 U1.1 U1.2
N$17: K3.8(COM) U1.3 U1.4
N$20: D2.1(K) J8.1 J8.2 K7.5(COIL_2)
N$21: D3.1(K) J9.1 J9.2 K7.2(COM)
N$22: K3.2(COIL_2) K7.4(NC)
N$23: J10.2 K6.8(COM)
N$25: J10.1 K6.5(NO)
N$27: D4.1(K) J12.2 K6.1(COIL_1)
N$29: J11.2 U5.3 U5.4
N$30: K4.4(NC) K5.3(NO) U5.1 U5.2
N$32: J11.1 K4.3(NO) K5.4(NC)
N$35: J14.2 K8.8(COM)
N$38: J14.1 K8.5(NO)
N$39: D6.1(K) J16.2 K8.1(COIL_1)
N$40: K10.4(NO) K10.6(COM)
N$41: K10.3(COM_(+)) U8.1 U8.2 U8.3
N$43: D7.1(K) J17.1 J17.2 K9.1(COIL_1)
N$45: H4.B2,25(MOUNT) U6.1 U6.2 U6.3
N$48: K9.8(COM) K10.8(COIL_2) U7.3 U7.4
N$49: J15.2 U7.1 U7.2
N$57: H3.B2,25(MOUNT) K10.5(NO_(-))
N$58: D8.1(K) J18.2 K11.1(COIL_1)
N$59: D10.1(K) J20.2 K15.1(COIL_1)
N$60: D11.1(K) J21.2 K13.1(COIL_1)
N$61: D12.1(K) J22.2 K14.1(COIL_1)
N$62: D9.1(K) J19.2 K12.1(COIL_1)
N$63: D13.1(K) J23.2 K16.1(COIL_1)
N$64: J24.2 U9.1 U9.2
N$65: J25.2 U10.1 U10.2
N$66: J26.2 U11.1 U11.2
N$67: J31.2 J34.2 J36.2
N$68: J31.1 J34.1 J36.1
N$69: J38.2 U12.3 U12.4
R1INT: H1.B2,25(MOUNT) J4.N.O. J40.1 J40.2 K3.5(NO) K5.2(COM) K9.5(NO) U2.1 U2.2
R1INT1: H7.B2,25(MOUNT)
R2VC+INT: J4.VC+ J6.1 J6.2 K11.8(COM)
R11VC+INT: D5.1(K) J13.2 K4.5(COIL_2) K5.1(COIL_1) K15.8(COM)
REV+INT: J29.2 K13.8(COM) U11.3 U11.4
Unconnected: J1.1 J2.1 J3.N.C. J4.N.C. J12.1 J13.1 J15.1 J16.1 J18.1 J19.1 J20.1 J21.1 J22.1 J23.1 J24.1 J25.1 J26.1 J27.1 J28.1 J29.1 K7.3(NO)

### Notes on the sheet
- PCB Schematic
- LEGENDS:
- Dotted boxes shows connections of Relays according to individual  functionalities
- 1
- 2
- Connectors with P.N 87427-0242 fixed on PCB and P.N 39-01-2020 female signal
  connectors wil connect on top to connect different signals  with PCB
- With purple color, names of signals which will be connected to Connectors are mentioned
- Those connectors with which nothing is mentioned to connect are not used for now for Prototype.
- On the PCB, Screw and nuts used to connect wires with the mounting holes
- +12V_PCB_KEYON
- KEY_ON signal
- 30A (GREEN) | R1 (ON CLICK) | R6 (CHG EN) | R2c (VAC.dSpace) | R9 (REV.dSpace)
- 12VBattGnd
- R2VC+INT
- +12VBatt
- Vacuum_Pump | +12VBatt
- 12VBattGnd
- +12VBatt | VAC_PWR signal
- 20A (YELLOW) | R2 (VAC.) | R12 (MPPTdSpace) | R10 (BRAKEdSpace)
- 3A (PURPLE)
- R11VC+IINT
- HVBat_DC12V+_Out signal
- DC12V+ for HV Battery | 2A (GREY) | R3 (HV BATT PWR) | R13 (BUZZERdSpace)
- R11c (PPAWLdSpace)
- ACCHG_12V signal
- R1INT
- Continue_Electric_12V+ for Inverter | 12VBattGnd
- R11/R11a (PPAWL)
- MPPT+INT
- 5A (BEIGE) | Inverter_PWR
- 12VBattGnd
- R4/R5 (INV. PWR)
- R1INT | Buzzer_out
- R1INT
- R7 (DC/DC EN)
- 12VBattGND
- +12VBatt | 10A (RED)
- For VMU Supply
- 1. Enable DC/DC
  2.+100V_PCB
- DC/DC_PWR signal
- VMU SUPPLY
- EMERGENCY
- 12V Bus_sense signal
- Connectors for VMU CAN Network
- Heater_PWR signal | 12V BUS SENSE
- CAN
- Liquid Heater
- Brake+INT
- 15A (HV)
- +100V_PCB
- 2A (GREY)
- MPPT SUPPLY | THROT./BRAKE +12V SUPPLY
- Liquid Heater Pump
- 2A (GREY)
- R8/R8a (HEATER)
  (HEATER PUMP)
- 3A (PURPLE)
- BRAKE LIGHTS
- BUZZER OUT
- 3A (PURPLE)
- REV. LIGHTS

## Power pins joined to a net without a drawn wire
P+: U$25.P$12(P+)
P-: U$25.P$13(P-)

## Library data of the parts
D1-D13 = AS1M-HF:AS1M-HF: Rectifiers AUTOMOTIVE RECTIFIER GEN PURP 1000V 1A SMA SMD General Purpose Rectifiers; DESCRIPTION: Rectifiers AUTOMOTIVE RECTIFIER GEN PURP 1000V 1A SMA SMD General Purpose Rectifiers; HEIGHT: 2.15mm; MANUFACTURER_NAME: Comchip Technology; MANUFACTURER_PART_NUMBER: AS1M-HF
DRIVING_-PROFILE_SWITCH S2 S4-S6 S10 = switch-omron:31-XX: OMRON SWITCH; MPN: B3F-3100; OC_FARNELL: 959704; OC_NEWARK: 36M3582
F1_(30A) F2_(20A) F4_(5A) F8_(2A) F9_(2A) F11_(450A)1 F12_(10A)2 F12_(15A) = special:FUSE: FUSE
H1 H1' H2 H2' H3 H3' H4 H4' H5 H5' H6 H6' H7 H8 = EVERGRIN_holes:MOUNT-PAD-ROUND: MOUNTING PAD, round
J1 J2 J5-J41 = 87427-0242:87427-0242: Headers & Wire Housings MINI-FIT JR. W-TO-B; ALLIED_NUMBER: 70374145; DESCRIPTION: Headers & Wire Housings MINI-FIT JR. W-TO-B; HEIGHT: 13.7mm; MANUFACTURER_NAME: Molex; MANUFACTURER_PART_NUMBER: 87427-0242; RS_PART_NUMBER: 6705887P; RS_PRICE-STOCK: http://uk.rs-online.com/web/p/products/6705887P
J3 J4 = VCF4-1000:VCF4-1000: Relay Socket; PCB; VTF Series; 1 Pole; Quick-Connect; w/o Grounding Provision Source: Datasheet; ALLIED_NUMBER: 70198724; DESCRIPTION: Relay Socket; PCB; VTF Series; 1 Pole; Quick-Connect; w/o Grounding Provision; HEIGHT: mm; MANUFACTURER_NAME: TE Connectivity; MANUFACTURER_PART_NUMBER: VCF4-1000; RS_PART_NUMBER: 2509255350; RS_PRICE-STOCK: http://uk.rs-online.com/web/p/products/2509255350
K1 K3 K6 K8 K9 K11-K16 = G6DN-1A_DC12:G6DN-1A_DC12: General Purpose Relays Source: Datasheet; ALLIED_NUMBER: 70788813; DESCRIPTION: General Purpose Relays; HEIGHT: 12.5mm; MANUFACTURER_NAME: Omron Electronics; MANUFACTURER_PART_NUMBER: G6DN-1A DC12; RS_PART_NUMBER: 2051950; RS_PRICE-STOCK: http://uk.rs-online.com/web/p/products/2051950
K2 = relay:G5L: RELAY 1 x switch, 10 A/120 V AC, 8 A/30 V ADC, Omron; OC_FARNELL: unknown; OC_NEWARK: unknown
K4 K5 K7 = G5Q-1-EU-DC12:G5Q-1-EU-DC12: Power Relay 12VDC 5(NO)/3(NC)DC/10(NO)/3(NC)AAC SPDT (20.3mm 10.3mm 15.8mm) THT Source: Datasheet; DESCRIPTION: Power Relay 12VDC 5(NO)/3(NC)DC/10(NO)/3(NC)AAC SPDT (20.3mm 10.3mm 15.8mm) THT; HEIGHT: 16.2mm; MANUFACTURER_NAME: Omron Electronics; MANUFACTURER_PART_NUMBER: G5Q-1-EU-DC12
K10 = G2RG-2A-X_DC12:G2RG-2A-X_DC12: General Purpose Relays 500VDC/10A high-voltage switching relay (2-pole wiring) Source: Datasheet; DESCRIPTION: General Purpose Relays 500VDC/10A high-voltage switching relay (2-pole wiring); HEIGHT: 29.5mm; MANUFACTURER_NAME: Omron Electronics; MANUFACTURER_PART_NUMBER: G2RG-2A-X DC12
MAIN_CONTACTOR1 PRESSURE_RELAY1 R1 R2 R2_C R3-R8 R8_A R22 = relay:APF30212A: Compliant with European standards 1a/1c 6A Slim power relays Source: Data sheet; OC_FARNELL: unknown
S1 S3 S7-S9 = switch-dil:DS01E: DIL/CODE SWITCH; OC_FARNELL: unknown; OC_NEWARK: unknown
U1 U5 U9-U12 = 3568-10:3568-10: FUSE SOCKET (RED) / BULK Source: Datasheet; ALLIED_NUMBER: 71172303; DESCRIPTION: FUSE SOCKET (RED) / BULK; HEIGHT: 7.5mm; MANUFACTURER_NAME: Keystone Electronics; MANUFACTURER_PART_NUMBER: 3568-10
U2-U4 U7 = 3568:3568: Fuse Holder 30A 500V 1 Circuit Blade Through Hole Source: Datasheet; DESCRIPTION: Fuse Holder 30A 500V 1 Circuit Blade Through Hole; HEIGHT: 7.5mm; MANUFACTURER_NAME: Keystone Electronics; MANUFACTURER_PART_NUMBER: 3568
U6 U8 = 0751.0506:0751.0506: Schurter 0751 Copper Alloy PCB Mount Fuse Clip for 10.3 x 85mm Source: Datasheet; ALLIED_NUMBER: 70255345; DESCRIPTION: Schurter 0751 Copper Alloy PCB Mount Fuse Clip for 10.3 x 85mm; HEIGHT: 20.7mm; MANUFACTURER_NAME: SCHURTER; MANUFACTURER_PART_NUMBER: 0751.0506; RS_PART_NUMBER: 8936991; RS_PRICE-STOCK: http://uk.rs-online.com/web/p/products/8936991
U$1 = EVERGRIN_Panda_G2:IGNITION_LOCK
U$2 = EVERGRIN_Panda_G2:EMERGENCY_BUTTON
U$3 U$4 U$27 = EVERGRIN_Panda_G2:VMU
U$14 = EVERGRIN_Panda_G2:INVERTER: Inverter
U$15 = EVERGRIN_Panda_G2:MOTOR: Motor
U$16 = EVERGRIN_Panda_G2:VACUUM_PUMP
U$19 = EVERGRIN_Panda_G2:DC/DC
U$20 = EVERGRIN_Panda_G2:LIQUID_HEATER: Liquid Heater
U$21 = EVERGRIN_Panda_G2:LIQUID_HEATER_PUMP: Liquid Heater Pump
U$22 = EVERGRIN_Panda_G2:12V_BATTERY: 12 V battery
U$23 = EVERGRIN_Panda_G2:ACC_PEDAL: Accelerator pedal
U$25 = EVERGRIN_Panda_G2:HV_BATTERY_BOX: HV battery box
U$26 = EVERGRIN_Panda_G2:1.8KW_BATTERY_CHARGER: 1.8 kW battery charger

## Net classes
0 default: width 0.254 mm, clearance 0.254 mm
1 CAN diff: width 1.219 mm, clearance 1 mm to class 0, clearance 1 mm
